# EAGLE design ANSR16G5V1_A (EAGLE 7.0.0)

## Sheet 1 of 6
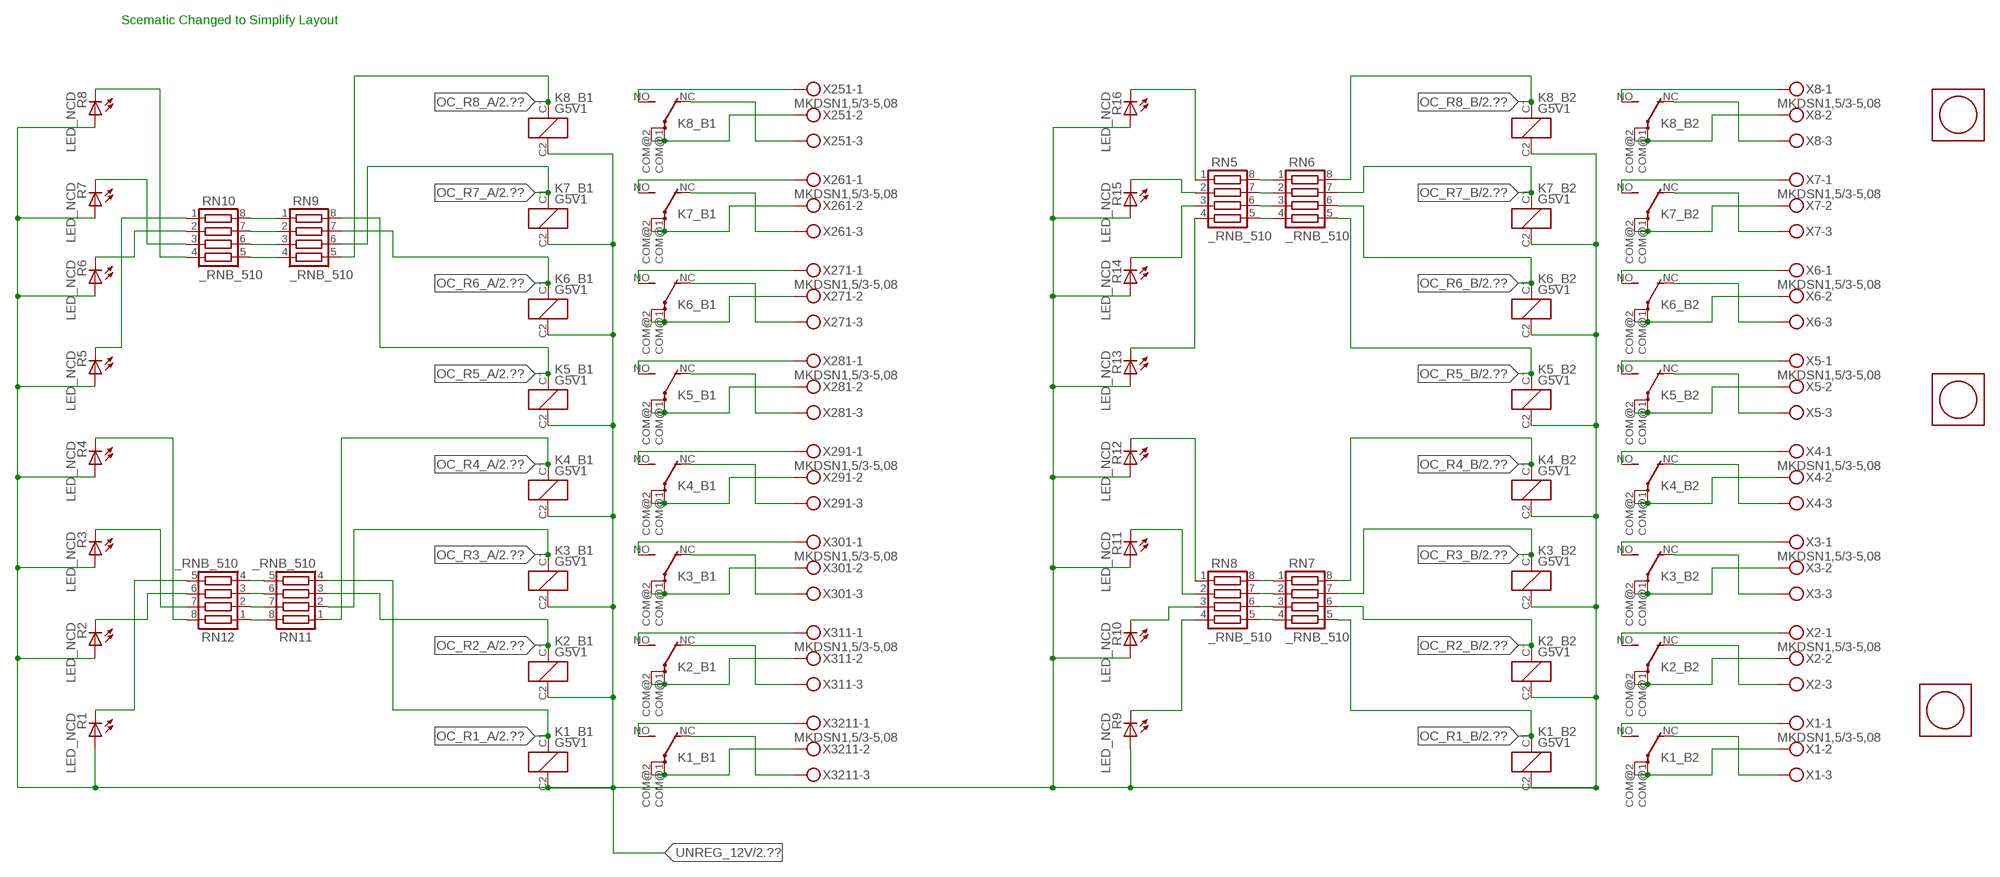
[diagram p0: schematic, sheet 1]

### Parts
K1_B1  G5V1  [G5V1]
K1_B2  G5V1  [G5V1]
K2_B1  G5V1  [G5V1]
K2_B2  G5V1  [G5V1]
K3_B1  G5V1  [G5V1]
K3_B2  G5V1  [G5V1]
K4_B1  G5V1  [G5V1]
K4_B2  G5V1  [G5V1]
K5_B1  G5V1  [G5V1]
K5_B2  G5V1  [G5V1]
K6_B1  G5V1  [G5V1]
K6_B2  G5V1  [G5V1]
K7_B1  G5V1  [G5V1]
K7_B2  G5V1  [G5V1]
K8_B1  G5V1  [G5V1]
K8_B2  G5V1  [G5V1]
R1  LED_NCD  [CHIPLED_0603]
R2  LED_NCD  [CHIPLED_0603]
R3  LED_NCD  [CHIPLED_0603]
R4  LED_NCD  [CHIPLED_0603]
R5  LED_NCD  [CHIPLED_0603]
R6  LED_NCD  [CHIPLED_0603]
R7  LED_NCD  [CHIPLED_0603]
R8  LED_NCD  [CHIPLED_0603]
R9  LED_NCD  [CHIPLED_0603]
R10  LED_NCD  [CHIPLED_0603]
R11  LED_NCD  [CHIPLED_0603]
R12  LED_NCD  [CHIPLED_0603]
R13  LED_NCD  [CHIPLED_0603]
R14  LED_NCD  [CHIPLED_0603]
R15  LED_NCD  [CHIPLED_0603]
R16  LED_NCD  [CHIPLED_0603]
RN5  _RNB_510  [RNB]
RN6  _RNB_510  [RNB]
RN7  _RNB_510  [RNB]
RN8  _RNB_510  [RNB]
RN9  _RNB_510  [RNB]
RN10  _RNB_510  [RNB]
RN11  _RNB_510  [RNB]
RN12  _RNB_510  [RNB]
U$1  PCB_MOUNTING_HOLE  [PCB_MOUNTING_HOLE]
U$2  PCB_MOUNTING_HOLE  [PCB_MOUNTING_HOLE]
U$3  PCB_MOUNTING_HOLE  [PCB_MOUNTING_HOLE]
X1  MKDSN1,5/3-5,08  [MKDSN1,5/3-5,08]
X2  MKDSN1,5/3-5,08  [MKDSN1,5/3-5,08]
X3  MKDSN1,5/3-5,08  [MKDSN1,5/3-5,08]
X4  MKDSN1,5/3-5,08  [MKDSN1,5/3-5,08]
X5  MKDSN1,5/3-5,08  [MKDSN1,5/3-5,08]
X6  MKDSN1,5/3-5,08  [MKDSN1,5/3-5,08]
X7  MKDSN1,5/3-5,08  [MKDSN1,5/3-5,08]
X8  MKDSN1,5/3-5,08  [MKDSN1,5/3-5,08]
X251  MKDSN1,5/3-5,08  [MKDSN1,5/3-5,08]
X261  MKDSN1,5/3-5,08  [MKDSN1,5/3-5,08]
X271  MKDSN1,5/3-5,08  [MKDSN1,5/3-5,08]
X281  MKDSN1,5/3-5,08  [MKDSN1,5/3-5,08]
X291  MKDSN1,5/3-5,08  [MKDSN1,5/3-5,08]
X301  MKDSN1,5/3-5,08  [MKDSN1,5/3-5,08]
X311  MKDSN1,5/3-5,08  [MKDSN1,5/3-5,08]
X3211  MKDSN1,5/3-5,08  [MKDSN1,5/3-5,08]

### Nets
N$1: K8_B2.COM@1(2:P) K8_B2.COM@2(2:P) X8.2
N$2: K8_B2.NC(2:O) X8.3
N$3: K8_B2.NO(2:S) X8.1
N$4: K7_B2.NO(2:S) X7.1
N$5: K6_B2.NO(2:S) X6.1
N$6: K7_B2.NC(2:O) X7.3
N$7: K7_B2.COM@1(2:P) K7_B2.COM@2(2:P) X7.2
N$8: K6_B2.NC(2:O) X6.3
N$10: K4_B2.NO(2:S) X4.1
N$11: K4_B2.NC(2:O) X4.3
N$12: K4_B2.COM@1(2:P) K4_B2.COM@2(2:P) X4.2
N$14: K6_B2.COM@1(2:P) K6_B2.COM@2(2:P) X6.2
N$33: K5_B2.NC(2:O) X5.3
N$34: K5_B2.COM@1(2:P) K5_B2.COM@2(2:P) X5.2
N$35: K5_B2.NO(2:S) X5.1
N$36: K3_B2.NO(2:S) X3.1
N$37: K3_B2.NC(2:O) X3.3
N$38: K3_B2.COM@1(2:P) K3_B2.COM@2(2:P) X3.2
N$39: K2_B2.NO(2:S) X2.1
N$40: K2_B2.NC(2:O) X2.3
N$41: K2_B2.COM@1(2:P) K2_B2.COM@2(2:P) X2.2
N$42: K1_B2.NO(2:S) X1.1
N$43: K1_B2.NC(2:O) X1.3
N$44: K1_B2.COM@1(2:P) K1_B2.COM@2(2:P) X1.2
N$203: K8_B1.COM@1(2:P) K8_B1.COM@2(2:P) X251.2
N$204: K8_B1.NC(2:O) X251.3
N$205: K8_B1.NO(2:S) X251.1
N$206: K7_B1.NO(2:S) X261.1
N$207: K6_B1.NO(2:S) X271.1
N$208: K7_B1.NC(2:O) X261.3
N$209: K7_B1.COM@1(2:P) K7_B1.COM@2(2:P) X261.2
N$210: K6_B1.NC(2:O) X271.3
N$211: K6_B1.COM@1(2:P) K6_B1.COM@2(2:P) X271.2
N$212: K5_B1.NC(2:O) X281.3
N$213: K5_B1.COM@1(2:P) K5_B1.COM@2(2:P) X281.2
N$214: K5_B1.NO(2:S) X281.1
N$215: K4_B1.NO(2:S) X291.1
N$216: K4_B1.NC(2:O) X291.3
N$217: K4_B1.COM@1(2:P) K4_B1.COM@2(2:P) X291.2
N$218: K3_B1.NO(2:S) X301.1
N$219: K3_B1.NC(2:O) X301.3
N$220: K3_B1.COM@1(2:P) K3_B1.COM@2(2:P) X301.2
N$221: K2_B1.NO(2:S) X311.1
N$222: K2_B1.NC(2:O) X311.3
N$223: K2_B1.COM@1(2:P) K2_B1.COM@2(2:P) X311.2
N$224: K1_B1.NO(2:S) X3211.1
N$225: K1_B1.NC(2:O) X3211.3
N$226: K1_B1.COM@1(2:P) K1_B1.COM@2(2:P) X3211.2
N$441: R16.C RN5.1
N$442: RN7.2 RN8.7
N$443: RN7.3 RN8.6
N$444: RN7.4 RN8.5
N$445: R15.C RN5.2
N$447: R13.C RN5.4
N$448: RN5.5 RN6.4
N$449: RN7.1 RN8.8
N$450: R12.C RN8.1
N$451: RN5.6 RN6.3
N$452: R11.C RN8.2
N$453: RN5.7 RN6.2
N$454: RN5.8 RN6.1
N$458: R14.C RN5.3
N$459: R10.C RN8.3
N$463: RN11.5 RN12.4
N$470: R9.C RN8.4
N$473: R1.C RN12.5
N$474: RN11.6 RN12.3
N$475: R2.C RN12.6
N$476: R3.C RN12.7
N$477: RN9.4 RN10.5
N$478: RN9.3 RN10.6
N$479: RN9.2 RN10.7
N$480: RN9.1 RN10.8
N$481: RN11.7 RN12.2
N$482: R5.C RN10.1
N$483: R4.C RN12.8
N$484: R7.C RN10.3
N$485: R8.C RN10.4
N$486: R6.C RN10.2
N$500: RN11.8 RN12.1
OC_R1_A: K1_B1.C1(1:C1) RN11.4 ; also sheet 2
OC_R1_B: K1_B2.C1(1:C1) RN7.5 ; also sheet 2
OC_R2_A: K2_B1.C1(1:C1) RN11.3 ; also sheet 2
OC_R2_B: K2_B2.C1(1:C1) RN7.6 ; also sheet 2
OC_R3_A: K3_B1.C1(1:C1) RN11.2 ; also sheet 2
OC_R3_B: K3_B2.C1(1:C1) RN7.7 ; also sheet 2
OC_R4_A: K4_B1.C1(1:C1) RN11.1 ; also sheet 2
OC_R4_B: K4_B2.C1(1:C1) RN7.8 ; also sheet 2
OC_R5_A: K5_B1.C1(1:C1) RN9.8 ; also sheet 2
OC_R5_B: K5_B2.C1(1:C1) RN6.5 ; also sheet 2
OC_R6_A: K6_B1.C1(1:C1) RN9.7 ; also sheet 2
OC_R6_B: K6_B2.C1(1:C1) RN6.6 ; also sheet 2
OC_R7_A: K7_B1.C1(1:C1) RN9.6 ; also sheet 2
OC_R7_B: K7_B2.C1(1:C1) RN6.7 ; also sheet 2
OC_R8_A: K8_B1.C1(1:C1) RN9.5 ; also sheet 2
OC_R8_B: K8_B2.C1(1:C1) RN6.8 ; also sheet 2
UNREG_12V: K1_B1.C2(1:C2) K1_B2.C2(1:C2) K2_B1.C2(1:C2) K2_B2.C2(1:C2) K3_B1.C2(1:C2) K3_B2.C2(1:C2) K4_B1.C2(1:C2) K4_B2.C2(1:C2) K5_B1.C2(1:C2) K5_B2.C2(1:C2) K6_B1.C2(1:C2) K6_B2.C2(1:C2) K7_B1.C2(1:C2) K7_B2.C2(1:C2) K8_B1.C2(1:C2) K8_B2.C2(1:C2) R1.A R2.A R3.A R4.A R5.A R6.A R7.A R8.A R9.A R10.A R11.A R12.A R13.A R14.A R15.A R16.A ; also sheet 2,3

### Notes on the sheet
- Scematic Changed to Simplify Layout

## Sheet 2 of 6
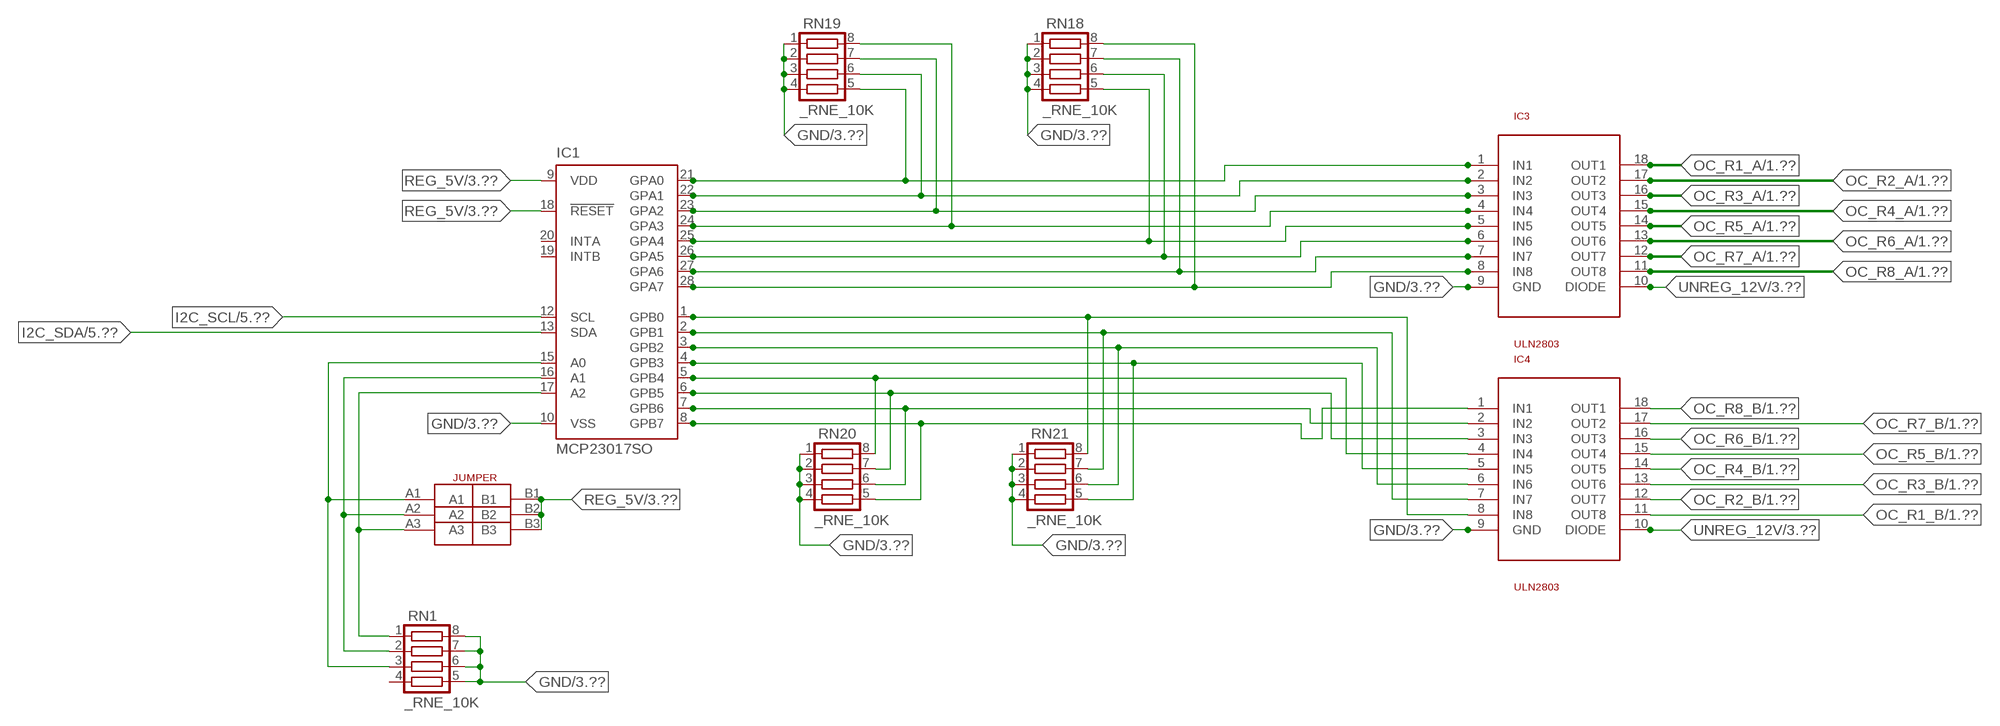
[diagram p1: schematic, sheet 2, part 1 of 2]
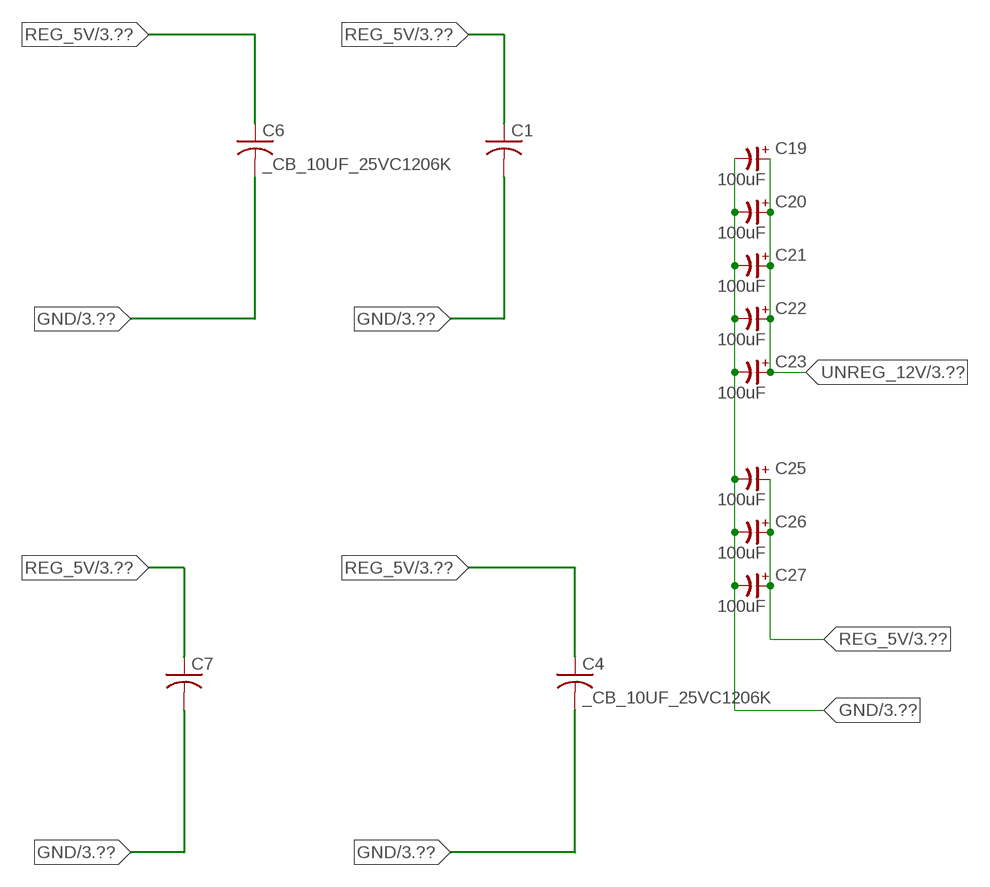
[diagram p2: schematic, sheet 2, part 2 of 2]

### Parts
C1  _CA_.10UF_50VC1206K  [_CA_.1UF_50V]
C4  _CB_10UF_25VC1206K  [_CB_10UF_25V]
C6  _CB_10UF_25VC1206K  [_CB_10UF_25V]
C7  _CA_.10UF_50VC1206K  [_CA_.1UF_50V]
C19  100uF  CP-E-025X060  [E-025X060]
C20  100uF  CP-E-025X060  [E-025X060]
C21  100uF  CP-E-025X060  [E-025X060]
C22  100uF  CP-E-025X060  [E-025X060]
C23  100uF  CP-E-025X060  [E-025X060]
C25  100uF  CP-E-025X060  [E-025X060]
C26  100uF  CP-E-025X060  [E-025X060]
C27  100uF  CP-E-025X060  [E-025X060]
IC1  MCP23017SO  [SO28W]
IC3  ULN2803  [SO18L]
IC4  ULN2803  [SO18L]
JP1  JUMPER_3X2  [JUMPER_3X2]
RN1  _RNE_10K  [RNE]
RN18  _RNE_10K  [RNE]
RN19  _RNE_10K  [RNE]
RN20  _RNE_10K  [RNE]
RN21  _RNE_10K  [RNE]

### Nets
GND: C1.2 C4.2 C6.2 C7.2 C19.- C20.- C21.- C22.- C23.- C25.- C26.- C27.- IC1.10(VSS) IC3.9(GND) IC4.9(GND) RN1.5 RN1.6 RN1.7 RN1.8 RN18.1 RN18.2 RN18.3 RN18.4 RN19.1 RN19.2 RN19.3 RN19.4 RN20.1 RN20.2 RN20.3 RN20.4 RN21.1 RN21.2 RN21.3 RN21.4 ; also sheet 3,4,5,6
I2C_SCL: IC1.12(SCL) ; also sheet 5,6
I2C_SDA: IC1.13(SDA) ; also sheet 5,6
N$78: IC1.15(A0) JP1.A1 RN1.3
N$405: IC1.21(GPA0) IC3.1(IN1) RN19.5
N$406: IC1.25(GPA4) IC3.5(IN5) RN18.5
N$407: IC1.26(GPA5) IC3.6(IN6) RN18.6
N$408: IC1.16(A1) JP1.A2 RN1.2
N$409: IC1.22(GPA1) IC3.2(IN2) RN19.6
N$410: IC1.23(GPA2) IC3.3(IN3) RN19.7
N$411: IC1.24(GPA3) IC3.4(IN4) RN19.8
N$416: IC1.1(GPB0) IC4.8(IN8) RN21.8
N$417: IC1.2(GPB1) IC4.7(IN7) RN21.7
N$418: IC1.3(GPB2) IC4.6(IN6) RN21.6
N$419: IC1.4(GPB3) IC4.5(IN5) RN21.5
N$420: IC1.5(GPB4) IC4.4(IN4) RN20.8
N$421: IC1.6(GPB5) IC4.3(IN3) RN20.7
N$422: IC1.7(GPB6) IC4.2(IN2) RN20.6
N$423: IC1.8(GPB7) IC4.1(IN1) RN20.5
N$498: IC1.17(A2) JP1.A3 RN1.1
N$525: IC1.27(GPA6) IC3.7(IN7) RN18.7
N$526: IC1.28(GPA7) IC3.8(IN8) RN18.8
OC_R1_A: IC3.18(OUT1) ; also sheet 1
OC_R1_B: IC4.11(OUT8) ; also sheet 1
OC_R2_A: IC3.17(OUT2) ; also sheet 1
OC_R2_B: IC4.12(OUT7) ; also sheet 1
OC_R3_A: IC3.16(OUT3) ; also sheet 1
OC_R3_B: IC4.13(OUT6) ; also sheet 1
OC_R4_A: IC3.15(OUT4) ; also sheet 1
OC_R4_B: IC4.14(OUT5) ; also sheet 1
OC_R5_A: IC3.14(OUT5) ; also sheet 1
OC_R5_B: IC4.15(OUT4) ; also sheet 1
OC_R6_A: IC3.13(OUT6) ; also sheet 1
OC_R6_B: IC4.16(OUT3) ; also sheet 1
OC_R7_A: IC3.12(OUT7) ; also sheet 1
OC_R7_B: IC4.17(OUT2) ; also sheet 1
OC_R8_A: IC3.11(OUT8) ; also sheet 1
OC_R8_B: IC4.18(OUT1) ; also sheet 1
REG_5V: C1.1 C4.1 C6.1 C7.1 C25.+ C26.+ C27.+ IC1.9(VDD) IC1.18(!RESET) JP1.B1 JP1.B2 JP1.B3 ; also sheet 3,4,5,6
UNREG_12V: C19.+ C20.+ C21.+ C22.+ C23.+ IC3.10(DIODE) IC4.10(DIODE) ; also sheet 1,3
Unconnected: IC1.19(INTB) IC1.20(INTA) RN1.4

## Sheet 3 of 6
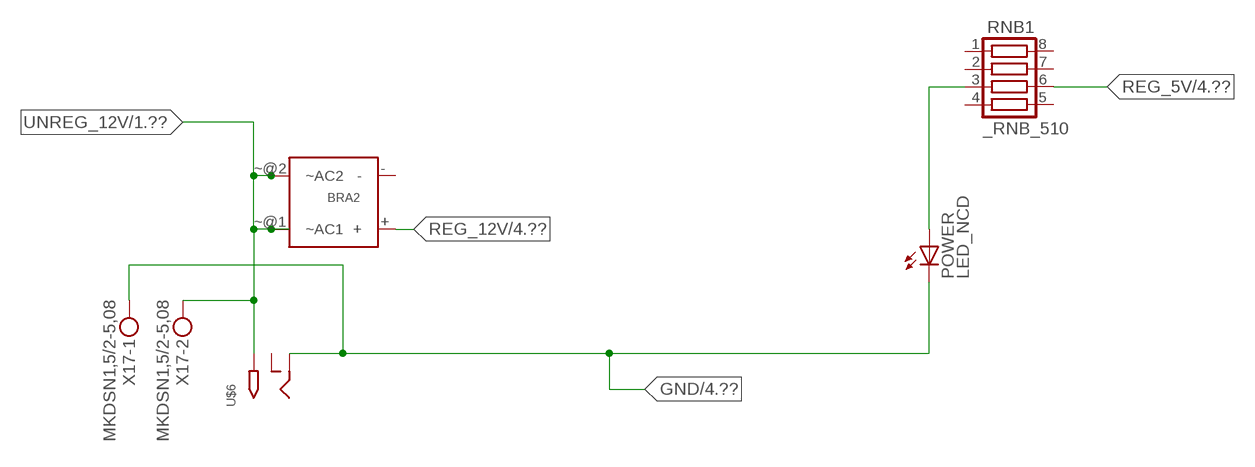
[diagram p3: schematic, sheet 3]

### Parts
BRA2  MB2S_  [MB2S]
POWER  LED_NCD  [CHIPLED_0603]
RNB1  _RNB_510  [RNB]
U$6  2.1MMJACK  [PJ-102A]
X17  MKDSN1,5/2-5,08  [MKDSN1,5/2-5,08]

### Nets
GND: POWER.C U$6.RING X17.1 ; also sheet 2,4,5,6
N$99: POWER.A RNB1.3
REG_5V: RNB1.6 ; also sheet 2,4,5,6
REG_12V: BRA2.+ ; also sheet 4
UNREG_12V: BRA2.~@1(~AC1) BRA2.~@2(~AC2) U$6.TIP X17.2 ; also sheet 1,2
Unconnected: BRA2.- RNB1.1 RNB1.2 RNB1.4 RNB1.5 RNB1.7 RNB1.8 U$6.RING_SW

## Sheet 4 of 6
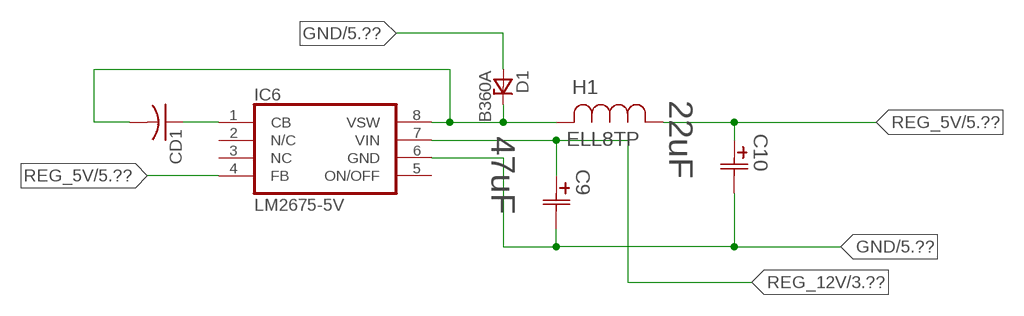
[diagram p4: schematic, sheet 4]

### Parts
C9  47uF  490-5463-6-NDCAP  [C2917(7343)-Y]
C10  22uF  490-5463-6-NDCAP  [C2917(7343)-Y]
CD1  _CD_10NF_50VC1206K  [_CD_10NF_50V]
D1  B360A  [DO214AC_ZENER]
H1  ELL8TP  [IND_ELL8TP]
IC6  LM2675-5V  LM2675  [SO-8]

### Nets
GND: C9.2(C2) C10.2(C2) D1.A IC6.6(GND) ; also sheet 2,3,5,6
N$100: CD1.2 D1.C H1.2 IC6.8(VSW)
N$101: CD1.1 IC6.1(CB)
REG_5V: C10.1(C1) H1.1 IC6.4(FB) ; also sheet 2,3,5,6
REG_12V: C9.1(C1) IC6.7(VIN) ; also sheet 3
Unconnected: IC6.2(N/C) IC6.5(ON/OFF)

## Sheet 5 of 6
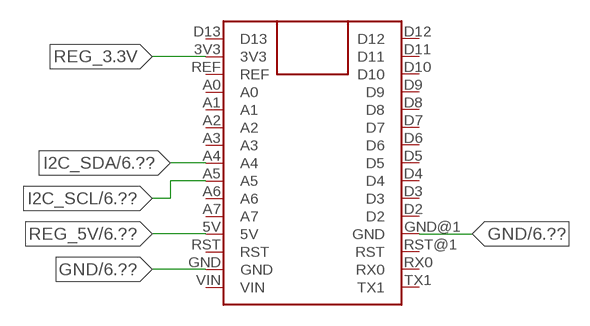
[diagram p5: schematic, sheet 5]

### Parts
FOR_NANO  ARDUINO_NANO  [ARDUINO_NANO]

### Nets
GND: FOR_NANO.GND FOR_NANO.GND@1(GND) ; also sheet 2,3,4,6
I2C_SCL: FOR_NANO.A5 ; also sheet 2,6
I2C_SDA: FOR_NANO.A4 ; also sheet 2,6
REG_3.3V: FOR_NANO.3V3
REG_5V: FOR_NANO.5V ; also sheet 2,3,4,6
Unconnected: FOR_NANO.A0 FOR_NANO.A1 FOR_NANO.A2 FOR_NANO.A3 FOR_NANO.A6 FOR_NANO.A7 FOR_NANO.D2 FOR_NANO.D3 FOR_NANO.D4 FOR_NANO.D5 FOR_NANO.D6 FOR_NANO.D7 FOR_NANO.D8 FOR_NANO.D9 FOR_NANO.D10 FOR_NANO.D11 FOR_NANO.D12 FOR_NANO.D13 FOR_NANO.REF FOR_NANO.RST FOR_NANO.RST@1(RST) FOR_NANO.RX0 FOR_NANO.TX1 FOR_NANO.VIN

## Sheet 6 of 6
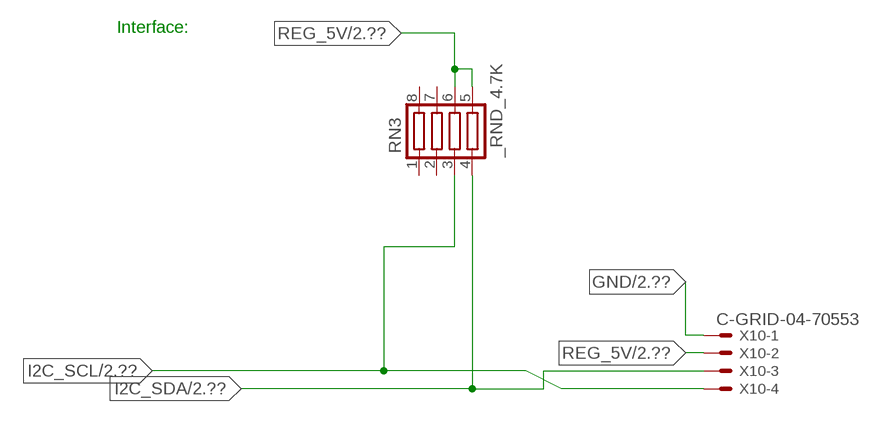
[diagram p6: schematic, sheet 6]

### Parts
RN3  _RND_4.7K  [RND]
X10  C-GRID-04-70553  [70553-04]

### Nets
GND: X10.1 ; also sheet 2,3,4,5
I2C_SCL: RN3.3 X10.4 ; also sheet 2,5
I2C_SDA: RN3.4 X10.3 ; also sheet 2,5
REG_5V: RN3.5 RN3.6 X10.2 ; also sheet 2,3,4,5
Unconnected: RN3.1 RN3.2 RN3.7 RN3.8

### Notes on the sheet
- Interface:

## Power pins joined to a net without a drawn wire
NC: IC6.3(NC)

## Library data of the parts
BRA2 = NCD_ULTIMATE_LIBRARY:MB2S: Bridge Rectifier BRA MB2S 200V 500ma Digikey MB2S-TPMSTR-ND/MB2S-TP
C1 C7 = NCD_ULTIMATE_LIBRARY:_CA_.10UF_50V: Capacitor .1uF SMT
C4 C6 = NCD_ULTIMATE_LIBRARY:_CB_10UF_25V: Capacitor 10uF SMT
C9 C10 = NCD_ULTIMATE_bhaskar:490-5463-6-ND: NCD CAP
C19-C23 C25-C27 = NCD_ULTIMATE_LIBRARY:CP-: Capacitors All Kinds POLARIZED CAP
CD1 = NCD_ULTIMATE_LIBRARY:_CD_10NF_50V: Capacitor 10nF SMT
D1 = NCD_ULTIMATE_bhaskar:B360A: NCD DIODE B350A/B360A
FOR_NANO = NCD_ULTIMATE_CONNECTORS:ARDUINO_NANO
H1 = NCD_ULTIMATE_bhaskar:ELL8TP: NCD coil
IC1 = NCD_ULTIMATE_LIBRARY:MCP23017: Semiconductor Port Expander I/O 16-Bit I2C http://ww1.microchip.com/downloads/en/DeviceDoc/21952a.pdf Source: http://ww1.microchip.com/downloads/en/DeviceDoc/21952a.pdf
IC3 IC4 = NCD_ULTIMATE_LIBRARY:ULN2803: Semiconductor 8 O.C. N-Channel Transistor Driver Digikey ULN2803AFWGCELTR-ND/ULN2803AFWG,C,EL
IC6 = NCD_ULTIMATE_bhaskar:LM2675: LM2675 NCD http://www.ti.com/lit/ds/symlink/lm2675.pdf
JP1 = NCD_ULTIMATE_CONNECTORS:JUMPER_3X2
K1_B1 K1_B2 K2_B1 K2_B2 K3_B1 K3_B2 K4_B1 K4_B2 K5_B1 K5_B2 K6_B1 K6_B2 K7_B1 K7_B2 K8_B1 K8_B2 = NCD_ULTIMATE_LIBRARY:G5V1: RELAY 1 x switch, 0.5 A/125 V AC, 1 A/24 V DC , Omron
POWER R1-R16 = NCD_ULTIMATE_bhaskar:LED_NCD
RN1 RN18-RN21 = NCD_ULTIMATE_LIBRARY:_RNE_10K: Resistor Array RNE SMT 10K x 4 Single Resistor Source: http://www.ctscorp.com/components/Datasheets/CTSChipArrayDs.pdf Digikey 742C083103JPTR-ND/742C083103JP; OC_FARNELL: unknown; OC_NEWARK: unknown
RN3 = NCD_ULTIMATE_LIBRARY:_RND_4.7K: Resistor Array RND SMT 4.7K x 4 Single Resistor Source: http://www.ctscorp.com/components/Datasheets/CTSChipArrayDs.pdf Digikey 742C083472JPTR-ND/742C083472JP; OC_FARNELL: unknown; OC_NEWARK: unknown
RN5-RN12 RNB1 = NCD_ULTIMATE_LIBRARY:_RNB_510: Resistor Array RNB SMT 510 x 4 Single Resistor Source: http://www.ctscorp.com/components/Datasheets/CTSChipArrayDs.pdf Digikey 742C083511JPTR-ND/ 742C083511JP; OC_FARNELL: unknown; OC_NEWARK: unknown
U$1-U$3 = NCD_ULTIMATE_CONNECTORS:PCB_MOUNTING_HOLE
U$6 = NCD_ULTIMATE_CONNECTORS:2.1MMJACK: 2.1mm x 5.5mm DC jack with internal switch. Digikey part #PJ-102A, 4UCON part #05537 By microbuilder.eu
X1-X8 X251 X261 X271 X281 X291 X301 X311 X3211 = NCD_ULTIMATE_CONNECTORS:MKDSN1,5/3-5,08: MKDSN 1,5/ 3-5,08 Printklemme Nennstrom: 13,5 A Nennspannung: 250 V Rastermaß: 5,08 mm Polzahl: 3 Anschlussart: Schraubanschluss Montage: Löten Anschlussrichtung Leiter/Platine: 0 ° Artikelnummer: 1729131 Source: http://eshop.phoenixcontact.com .. 1729131.pdf
X10 = NCD_ULTIMATE_CONNECTORS:C-GRID-04: CONNECTOR 4-Pos I2C wire to board 2.54 mm (0.100") pitch header Digikey WM1342-ND/0015912045; OC_FARNELL: unknown; OC_NEWARK: unknown
X17 = NCD_ULTIMATE_CONNECTORS:MKDSN1,5/2-5,08: MKDSN 1,5/ 2-5,08 Printklemme

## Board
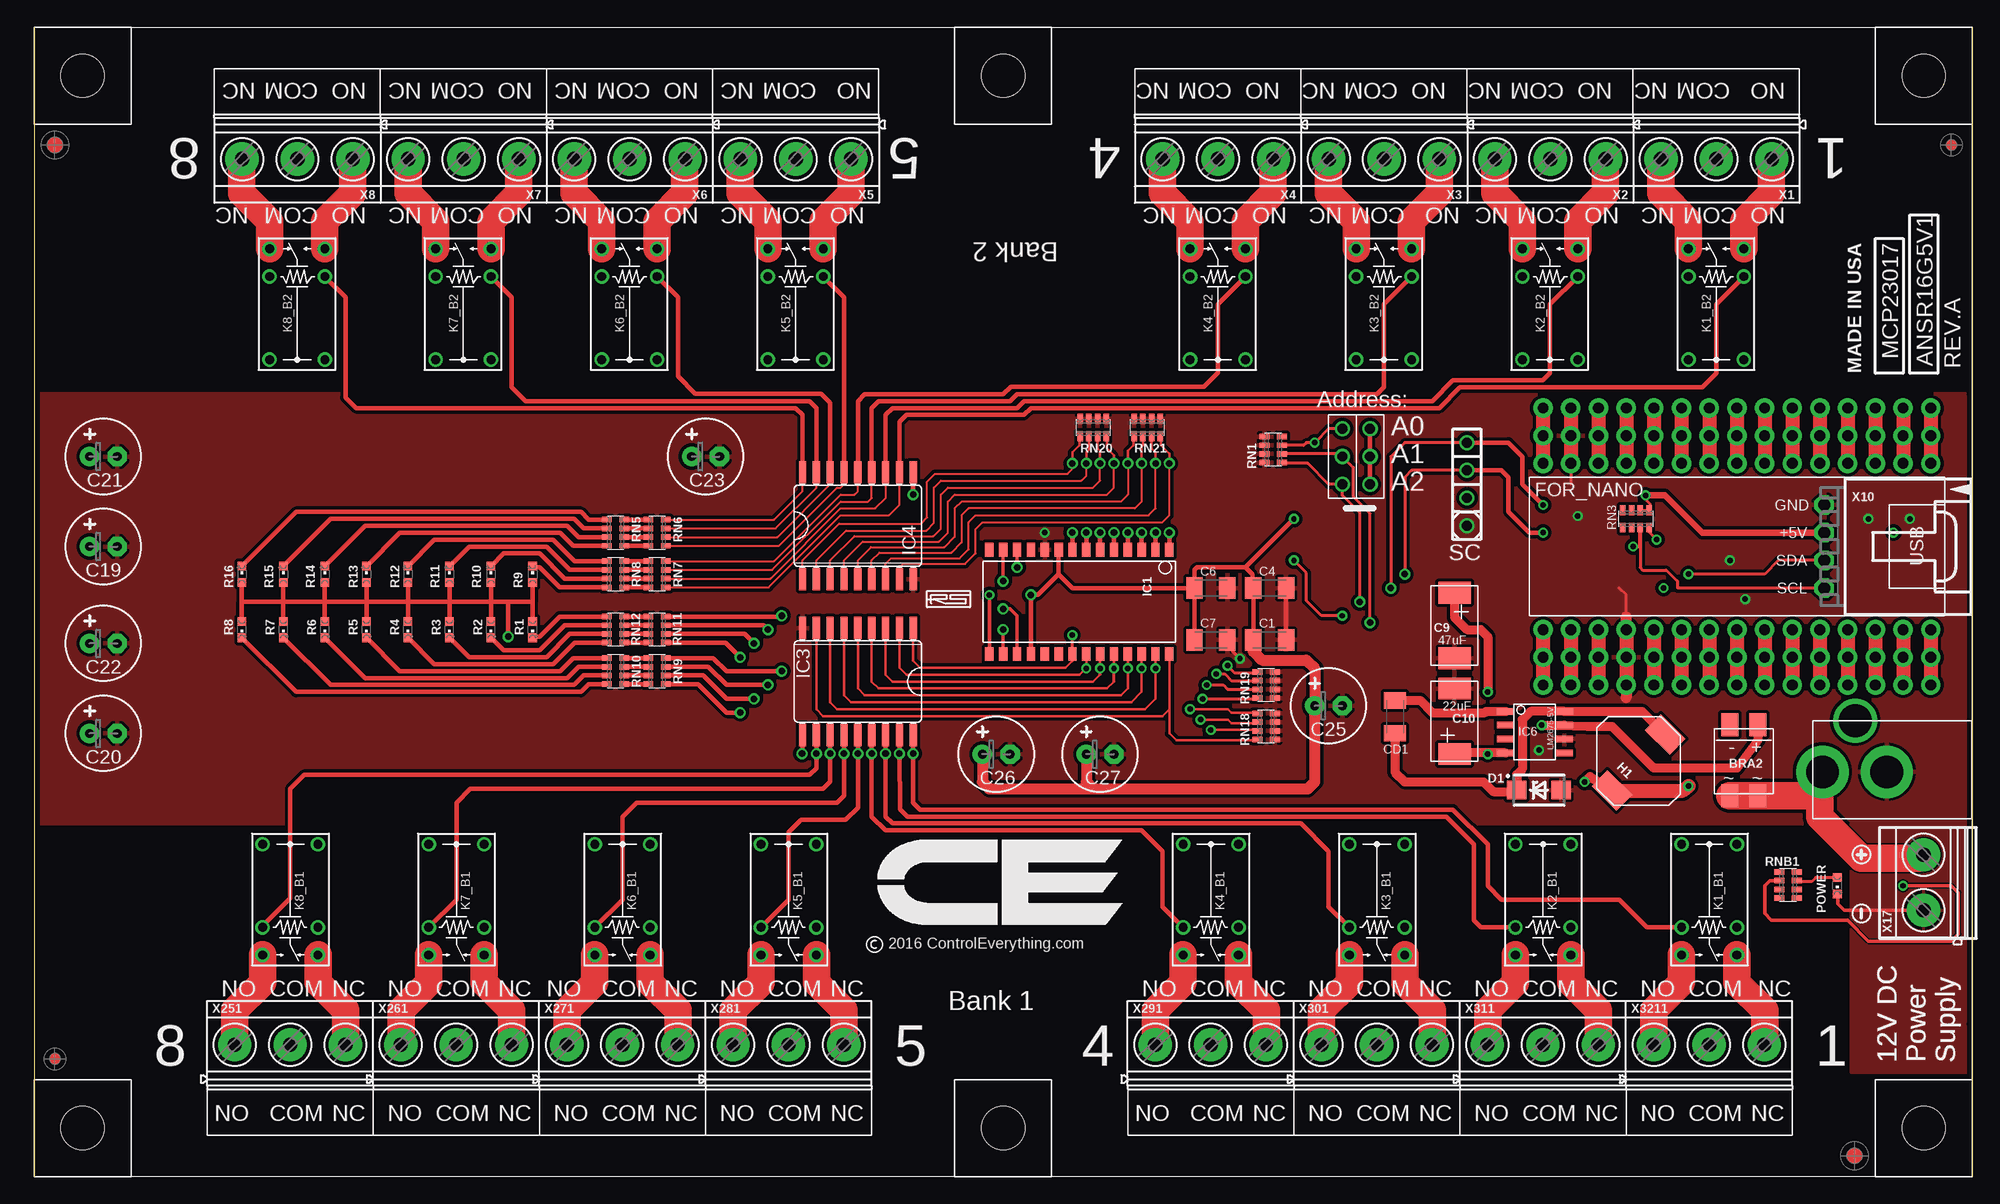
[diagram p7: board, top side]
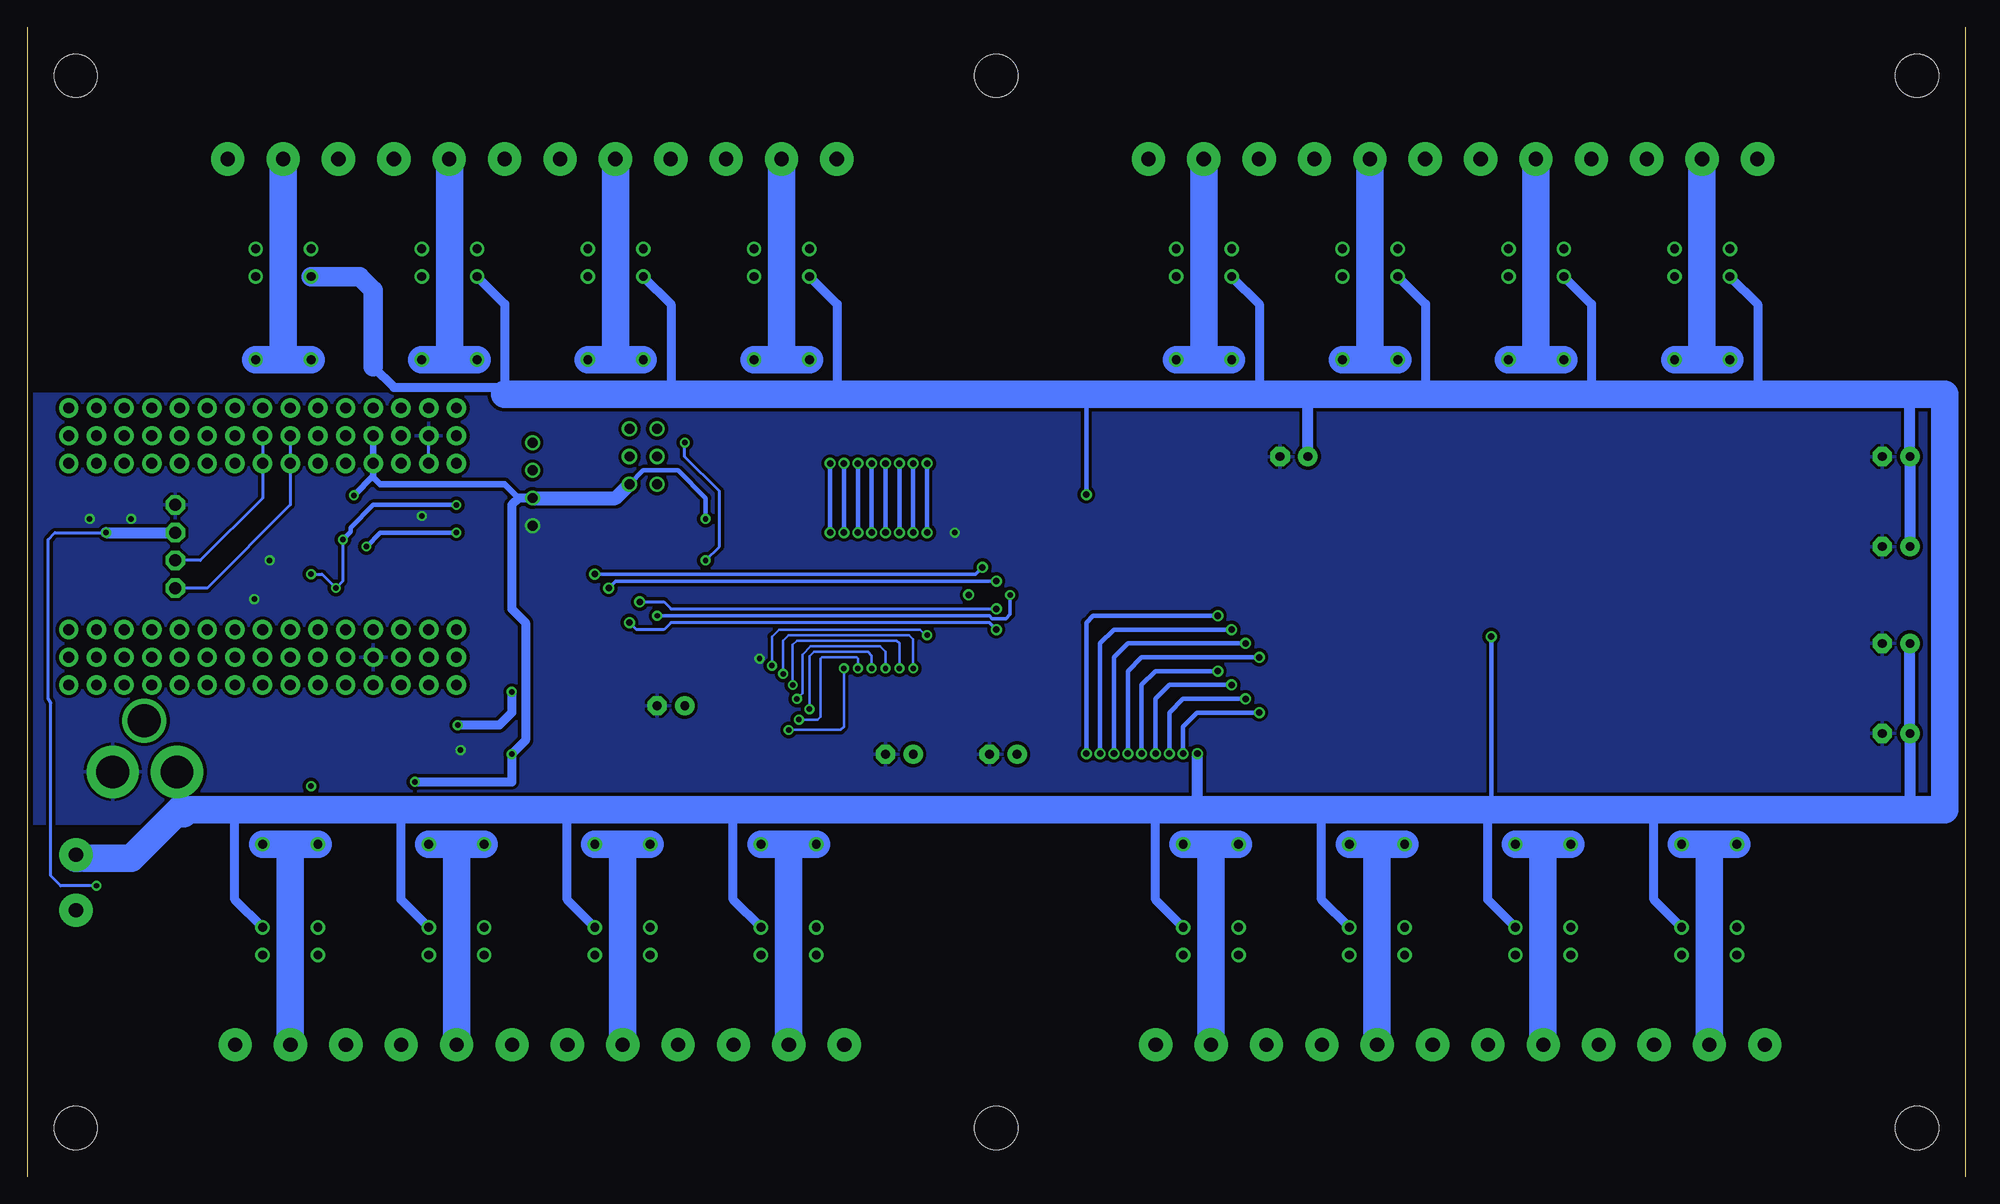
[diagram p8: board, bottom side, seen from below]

Size 177.8 x 105.42 mm. Coordinates in mm from the lower left corner, seen from the top.
Outline: 177.78,105.42 177.78,0
Outline: 0,105.42 0,0.01
Outline: 177.8,71.77 177.8,13.98
Copper layers (1*16): Top 0.035mm / dielectric 1.5mm / Bottom 0.035mm
Design rules "default *": minimum track width 6mil, minimum drill 12mil, track to track 5mil, track to pad 5mil, pad to pad 5mil, via to via 5mil, smd to smd 5mil, copper to edge 20mil, drill to drill 8mil, minimum pad ring 10mil, minimum via ring 8mil, stop-mask expansion 4mil, vias tented up to drill 0mil, thermal gap 10mil

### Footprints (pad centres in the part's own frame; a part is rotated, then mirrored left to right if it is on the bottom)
MB2S = smd 1.55 x 2.1: + 0,-6.5; - 2.54,-6.5; ~@1 0,0; ~@2 2.54,0
_CA_.1UF_50V = smd 1.5 x 2: 1 -1.5,0; 2 1.5,0
_CB_10UF_25V = smd 1.5 x 2: 1 -1.5,0; 2 1.5,0
C2917(7343)-Y = smd 2 x 3: 1 -3,0; 2 3,0
E-025X060 = drill 0.813 pad 1.778: + -1.27,0 | drill 0.813 pad 1.778 octagon: - 1.27,0
_CD_10NF_50V = smd 1.5 x 2: 1 -1.5,0; 2 1.5,0
DO214AC_ZENER = smd 1.8 x 1.7: A 2.05,0; C -2.05,0
ARDUINO_NANO = drill 1 pad 1.778: 3V1 -2.54,-2.54; 3V3 0,-2.54; 5V 0,-27.94; 5V1 -2.54,-27.94; A0 0,-7.62; A1 0,-10.16; A2 0,-12.7; A3 0,-15.24; A4 0,-17.78; A5 0,-20.32; A6 0,-22.86; A7 0,-25.4; A8 -2.54,-7.62; A9 -2.54,-10.16; A10 -2.54,-12.7; A11 -2.54,-15.24; A12 -2.54,-17.78; A13 -2.54,-20.32; A14 -2.54,-22.86; A15 -2.54,-25.4; D1 -2.54,0; D2 20.32,-25.4; D3 20.32,-22.86; D4 20.32,-20.32; D5 20.32,-17.78; D6 20.32,-15.24; D7 20.32,-12.7; D8 20.32,-10.16; D9 20.32,-7.62; D10 20.32,-5.08; D11 20.32,-2.54; D12 20.32,0; D13 0,0; D14 22.86,0; D15 22.86,-2.54; D16 22.86,-5.08; D17 22.86,-7.62; D18 22.86,-10.16; D19 22.86,-12.7; D20 22.86,-15.24; D21 22.86,-17.78; D22 22.86,-20.32; D23 22.86,-22.86; D24 22.86,-25.4; GND 0,-33.02; GND1 -2.54,-33.02; GND@1 20.32,-27.94; GND@2 22.86,-27.94; P$16 2.54,0; P$17 2.54,-2.54; P$18 2.54,-5.08; P$19 2.54,-7.62; P$20 2.54,-10.16; P$21 2.54,-12.7; P$22 2.54,-15.24; P$23 2.54,-17.78; P$24 2.54,-20.32; P$25 2.54,-22.86; P$26 2.54,-25.4; P$27 2.54,-27.94; P$28 2.54,-30.48; P$29 2.54,-33.02; P$30 2.54,-35.56; P$31 17.78,0; P$32 17.78,-2.54; P$33 17.78,-5.08; P$34 17.78,-7.62; P$35 17.78,-10.16; P$36 17.78,-12.7; P$37 17.78,-15.24; P$38 17.78,-17.78; P$39 17.78,-20.32; P$40 17.78,-22.86; P$41 17.78,-25.4; P$42 17.78,-27.94; P$43 17.78,-30.48; P$44 17.78,-33.02; P$45 17.78,-35.56; REF 0,-5.08; REF1 -2.54,-5.08; RST 0,-30.48; RST1 -2.54,-30.48; RST@1 20.32,-30.48; RST@2 22.86,-30.48; RX0 20.32,-33.02; RX1 22.86,-33.02; TX1 20.32,-35.56; TX2 22.86,-35.56; VIN 0,-35.56; VIN1 -2.54,-35.56
IND_ELL8TP = smd 2.054 x 3.2 rotated 45: 1 -2.442,-2.696; 2 2.442,2.442
SO28W = smd 0.762 x 1.27: 1 -7.62,-4.78; 2 -6.35,-4.78; 3 -5.08,-4.78; 4 -3.81,-4.78; 5 -2.54,-4.78; 6 -1.27,-4.78; 7 0,-4.78; 8 1.27,-4.78; 9 2.54,-4.78; 10 3.81,-4.78; 11 5.08,-4.78; 12 6.35,-4.78; 13 7.62,-4.78; 14 8.89,-4.78; 15 8.89,4.78; 16 7.62,4.78; 17 6.35,4.78; 18 5.08,4.78; 19 3.81,4.78; 20 2.54,4.78; 21 1.27,4.78; 22 0,4.78; 23 -1.27,4.78; 24 -2.54,4.78; 25 -3.81,4.78; 26 -5.08,4.78; 27 -6.35,4.78; 28 -7.62,4.78
SO18L = smd 0.66 x 2.032: 1 -5.08,-4.902; 2 -3.81,-4.902; 3 -2.54,-4.902; 4 -1.27,-4.902; 5 0,-4.902; 6 1.27,-4.902; 7 2.54,-4.902; 8 3.81,-4.902; 9 5.08,-4.902; 10 5.08,4.902; 11 3.81,4.902; 12 2.54,4.902; 13 1.27,4.902; 14 0,4.902; 15 -1.27,4.902; 16 -2.54,4.902; 17 -3.81,4.902; 18 -5.08,4.902
SO-8 = smd 0.6 x 1.55: 1 -1.905,-2.69; 2 -0.635,-2.69; 3 0.635,-2.69; 4 1.905,-2.69; 5 1.905,2.71; 6 0.635,2.71; 7 -0.635,2.71; 8 -1.905,2.71
JUMPER_3X2 = drill 0.9: A1 0,5.08; A2 0,2.54; A3 0,0; B1 2.54,5.08; B2 2.54,2.54; B3 2.54,0
G5V1 = drill 0.813: C1 -2.54,2.54; C2 -2.54,-2.54; COM@1 5.08,-2.54; COM@2 5.08,2.54; NC -5.08,-2.54; NO -5.08,2.54
CHIPLED_0603 = smd 0.8 x 0.8: A 0,-0.75; C 0,0.75
RNE = smd 0.5 x 0.9: 1 -1.2,-0.8; 2 -0.4,-0.8; 3 0.4,-0.8; 4 1.2,-0.8; 5 1.2,0.8; 6 0.4,0.8; 7 -0.4,0.8; 8 -1.2,0.8
RND = smd 0.5 x 0.9: 1 -1.2,-0.8; 2 -0.4,-0.8; 3 0.4,-0.8; 4 1.2,-0.8; 5 1.2,0.8; 6 0.4,0.8; 7 -0.4,0.8; 8 -1.2,0.8
RNB = smd 0.5 x 0.9: 1 -1.2,-0.8; 2 -0.4,-0.8; 3 0.4,-0.8; 4 1.2,-0.8; 5 1.2,0.8; 6 0.4,0.8; 7 -0.4,0.8; 8 -1.2,0.8
PCB_MOUNTING_HOLE = hole 3.962: 4.445,4.445
PJ-102A = drill 3 pad 4.8: RING 0.1,-3.39; TIP 0.1,-9.29 | drill 3 pad 3.251: RING_SW -4.6,-6.29
MKDSN1,5/3-5,08 = drill 1.3 pad 3.048: 1 -7.641,0.025; 2 -2.561,0.025; 3 2.519,0.025
70553-04 = drill 1.1 pad 1.778 octagon: 1 -3.81,-7.62; 2 -1.27,-7.62; 3 1.27,-7.62; 4 3.81,-7.62
MKDSN1,5/2-5,08 = drill 1.3 pad 3.048: 1 -2.561,0.025; 2 2.519,0.025

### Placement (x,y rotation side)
BRA2  158.12,34.94 180 top
C1  113.35,49.23 0 top
C4  113.35,53.99 0 top
C6  107.95,53.99 0 top
C7  107.95,49.23 0 top
C9  130.3,50.56 270 top
C10  130.3,41.77 90 top
C19  6.35,57.8 0 top
C20  6.35,40.65 0 top
C21  6.35,66.05 0 top
C22  6.35,48.91 0 top
C23  61.59,66.05 0 top
C25  118.75,43.19 0 top
C26  88.27,38.75 0 top
C27  97.79,38.75 0 top
CD1  124.84,42.18 270 top
D1  138.05,35.45 0 top
FOR_NANO  173.99,67.96 270 top
H1  147.19,38.11 0 top
IC1  96.52,52.72 180 top
IC3  75.56,45.42 180 top
IC4  75.56,59.7 0 top
IC6  137.67,40.78 270 top
JP1  120.02,63.51 0 top
K1_B1  153.67,25.41 90 top
K1_B2  154.31,80.02 270 top
K2_B1  138.43,25.41 90 top
K2_B2  139.06,80.02 270 top
K3_B1  123.19,25.41 90 top
K3_B2  123.83,80.02 270 top
K4_B1  107.95,25.41 90 top
K4_B2  108.58,80.02 270 top
K5_B1  69.22,25.41 90 top
K5_B2  69.85,80.02 270 top
K6_B1  53.98,25.41 90 top
K6_B2  54.61,80.02 270 top
K7_B1  38.73,25.41 90 top
K7_B2  39.37,80.02 270 top
K8_B1  23.5,25.41 90 top
K8_B2  24.13,80.02 270 top
POWER  165.42,26.68 180 top
R1  45.72,50.18 180 top
R2  41.91,50.18 180 top
R3  38.1,50.18 180 top
R4  34.29,50.18 180 top
R5  30.48,50.18 180 top
R6  26.67,50.18 180 top
R7  22.86,50.18 180 top
R8  19.05,50.18 180 top
R9  45.72,55.26 0 top
R10  41.91,55.26 0 top
R11  38.1,55.26 0 top
R12  34.29,55.26 0 top
R13  30.48,55.26 0 top
R14  26.67,55.26 0 top
R15  22.86,55.26 0 top
R16  19.05,55.26 0 top
RN1  113.67,66.69 90 top
RN3  146.94,60.34 0 top
RN5  53.34,59.07 270 top
RN6  57.15,59.07 270 top
RN7  57.15,55.26 270 top
RN8  53.34,55.26 270 top
RN9  57.15,46.37 270 top
RN10  53.34,46.37 270 top
RN11  57.15,50.18 90 top
RN12  53.34,50.18 90 top
RN18  113.03,41.29 90 top
RN19  113.03,45.1 90 top
RN20  97.16,68.72 180 top
RN21  102.11,68.72 180 top
RNB1  160.91,26.75 90 top
U$1  93.34,96.53 90 top
U$2  8.89,96.53 90 top
U$3  177.8,96.53 90 top
U$5  PCB_MOUNTING_HOLE  [PCB_MOUNTING_HOLE]  0,8.9 270 top
U$6  173.35,37.22 270 top
U$8  [ICON_MINUS]  167.64,24.14 90 top
U$9  PCB_MOUNTING_HOLE  [PCB_MOUNTING_HOLE]  8.89,96.53 90 top
U$10  PCB_MOUNTING_HOLE  [PCB_MOUNTING_HOLE]  84.45,8.9 270 top
U$11  PCB_MOUNTING_HOLE  [PCB_MOUNTING_HOLE]  168.91,8.9 270 top
U$12  PCB_MOUNTING_HOLE  [PCB_MOUNTING_HOLE]  0,8.9 270 top
U$13  [ICON_PLUS]  167.64,29.54 0 top
U$15  [VISION_REF15]  167,1.92 90 top
U$17  [ICON_MINUS]  167.64,24.14 90 top
U$18  [VISION_REF10]  175.9,94.63 90 top
U$19  [ICON_PLUS]  167.64,29.54 0 top
U$21  [ICON_USA]  167.64,73.67 90 top
U$22  [ICON_MINUS]  167.64,24.14 90 top
U$23  [VISION_REF15]  1.91,94.63 90 top
U$24  [ICON_PLUS]  167.64,29.54 0 top
U$28  [VISION_REF10]  1.91,10.81 90 top
X1  151.76,93.36 180 top
X2  136.53,93.36 180 top
X3  121.28,93.36 180 top
X4  106.05,93.36 180 top
X5  67.31,93.36 180 top
X6  52.07,93.36 180 top
X7  36.83,93.36 180 top
X8  21.59,93.36 180 top
X10  171.83,57.8 270 top
X17  173.35,27 90 top
X251  26.04,12.08 0 top
X261  41.27,12.08 0 top
X271  56.52,12.08 0 top
X281  71.75,12.08 0 top
X291  110.49,12.08 0 top
X301  125.73,12.08 0 top
X311  140.97,12.08 0 top
X3211  156.21,12.08 0 top

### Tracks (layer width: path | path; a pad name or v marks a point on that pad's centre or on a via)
GND  (via drill 0.5, 0.9)
  Top 0.254: 146.05,51.32 146.05,53.35 145.41,53.99 | FOR_NANO.GND@1 146.05,46.37 | 140.97,70.5 140.97,63.51
  Top 0.305: v110.62,47.51 109.22,48.91 109.22,49 C7.2 | X17.1 166.07,24.44 165.48,25.03 165.48,25.87 POWER.C
  Top 0.406: C1.2 C4.2
  Top 1.016: X10.1 164.06,61.61 | 146.05,43.95 146.05,50.18 146.05,51.32
  Bottom 0.254: 140.97,65.42 FOR_NANO.GND
  other vias: 92.71,59.07 131.44,59.7 168.28,60.34 141.6,60.59 172.09,60.34 155.57,56.53 156.97,52.97 138.05,39.13
  pour Top (isolate 0.305): -7.62,32.4 -7.62,71.77 178.12,71.77 178.12,32.4
  pour Top (isolate 0.305): 178.12,20.33 166.69,20.33 166.69,32.4 178.12,32.4
  pour Bottom (isolate 0.305): -4.45,32.4 -4.45,71.77 177.8,71.77 177.8,32.4
  pour Top (isolate 0.305): 177.48,9.54 166.69,9.54 166.69,32.4 177.48,32.4
  pour Top: 177.48,9.54 166.69,9.54 166.69,32.4 177.48,32.4
I2C_SCL  (via drill 0.5, 0.6, 0.9)
  Top 0.254: v131.44,64.78 126.36,64.78 125.73,64.15 v125.73,55.26 | X10.4 150.75,53.99 150.75,54.62 149.73,55.64 147.57,55.64 147.34,55.87 RN3.3 147.32,59.52 147.32,57.8 v146.69,57.8
  Top 0.305: v90.17,55.89 IC1.12
  Top 0.406: v131.44,64.78 134.62,64.78 135.25,64.15 135.25,60.97 137.16,59.07 v138.43,59.07
  Bottom 0.254: FOR_NANO.A5 153.67,61.61 161.29,53.99 X10.4
  Bottom 0.305: v125.73,55.26 90.81,55.26 v90.17,55.89
  Bottom 0.406: v138.43,59.07 145.41,59.07 v146.69,57.8
I2C_SDA  (via drill 0.5, 0.6, 0.9)
  Top 0.254: v131.44,67.32 125.73,67.32 124.46,66.05 v124.46,53.99 | RN3.4 148.14,59.14 v148.84,58.43 | 149.47,53.98 v149.48,53.99 | X10.3 160.02,56.53 158.75,55.26 v151.76,55.26
  Top 0.305: v88.9,54.62 IC1.13
  Top 0.406: v131.44,67.32 135.25,67.32 136.53,66.05 136.53,63.51 v138.43,61.61
  Bottom 0.254: v148.84,58.43 148.84,54.62 v149.48,53.99 150.75,55.26 v151.76,55.26 | FOR_NANO.A4 156.21,62.24 161.93,56.53 X10.3
  Bottom 0.305: v88.9,54.62 123.83,54.62 v124.46,53.99
  Bottom 0.406: v138.43,61.61 146.07,61.61 RN3.4 148.14,59.14 v148.84,58.43
N$1
  Bottom 2.54: K8_B2.COM@2 24.13,74.94 | 24.13,74.94 K8_B2.COM@1 | X8.2 24.15,74.96 24.13,74.94
N$2
  Top 2.54: K8_B2.NC 21.59,87.64 19.05,90.18 19.05,93.31 X8.3
N$3
  Top 2.54: K8_B2.NO 26.67,87.64 29.21,90.18 29.21,93.31 X8.1
N$4
  Top 2.54: K7_B2.NO 41.91,87.64 44.45,90.18 44.45,93.31 X7.1
N$5
  Top 2.54: K6_B2.NO 57.15,87.64 59.69,90.18 59.69,93.31 X6.1
N$6
  Top 2.54: K7_B2.NC 36.83,87.64 34.29,90.18 34.29,93.31 X7.3
N$7
  Bottom 2.54: K7_B2.COM@2 39.37,74.94 | 39.37,74.94 K7_B2.COM@1 | X7.2 39.39,74.96 39.37,74.94
N$8
  Top 2.54: K6_B2.NC 52.07,87.64 49.53,90.18 49.53,93.31 X6.3
N$10
  Top 2.54: K4_B2.NO 111.12,87.64 113.67,90.18 113.67,93.31 X4.1
N$11
  Top 2.54: K4_B2.NC 106.05,87.64 103.5,90.18 103.5,93.31 X4.3
N$12
  Bottom 2.54: K4_B2.COM@2 108.58,74.94 | 108.58,74.94 K4_B2.COM@1 | X4.2 108.61,74.96 108.58,74.94
N$14
  Bottom 2.54: K6_B2.COM@2 54.61,74.94 | 54.61,74.94 K6_B2.COM@1 | X6.2 54.63,74.96 54.61,74.94
N$33
  Top 2.54: K5_B2.NC 67.31,87.64 64.77,90.18 64.77,93.31 X5.3
N$34
  Bottom 2.54: K5_B2.COM@2 69.85,74.94 | 69.85,74.94 K5_B2.COM@1 | X5.2 69.87,74.96 69.85,74.94
N$35
  Top 2.54: K5_B2.NO 72.39,87.64 74.93,90.18 74.93,93.31 X5.1
N$36
  Top 2.54: K3_B2.NO 126.36,87.64 128.91,90.18 128.91,93.31 X3.1
N$37
  Top 2.54: K3_B2.NC 121.28,87.64 118.75,90.18 118.75,93.31 X3.3
N$38
  Bottom 2.54: 123.83,74.94 K3_B2.COM@1 | K3_B2.COM@2 123.83,74.94 | 123.83,74.94 123.83,93.31 X3.2
N$39
  Top 2.54: K2_B2.NO 141.6,87.64 144.15,90.18 144.15,93.31 X2.1
N$40
  Top 2.54: K2_B2.NC 136.53,87.64 133.99,90.18 133.99,93.31 X2.3
N$41
  Bottom 2.54: 139.06,74.94 K2_B2.COM@1 | K2_B2.COM@2 139.06,74.94 | 139.06,74.94 139.06,93.31 X2.2
N$42
  Top 2.54: K1_B2.NO 156.84,87.64 159.38,90.18 159.38,93.31 X1.1
N$43
  Top 2.54: K1_B2.NC 151.76,87.64 149.22,90.18 149.22,93.31 X1.3
N$44
  Bottom 2.54: K1_B2.COM@1 154.31,74.94 | K1_B2.COM@2 154.31,74.94 | 154.31,74.94 154.31,93.31 X1.2
N$78  (via drill 0.5)
  Top 0.254: v120.02,51.45 118.11,51.45 116.71,52.84 116.71,55.38 v115.57,56.53 | 114.48,67.07 116.46,67.07 116.71,67.32 v117.47,67.32 118.75,68.59 JP1.A1
  Top 0.305: IC1.15 v87.63,53.35 | 114.48,67.07 RN1.3
  Bottom 0.254: v115.57,56.53 114.3,57.8 114.3,62.88 117.47,66.05 v117.47,67.32
  Bottom 0.305: v87.63,53.35 87.63,51.57 88.01,51.19 89.28,51.19 89.53,51.45 v120.02,51.45
N$99
  Top 0.254: POWER.A 163.44,27.43 163.07,27.06 161.79,27.06 RNB1.3
  Top 0.406: 161.75,27.19 RNB1.3
N$100
  Top 0.813: 139.06,42.68 IC6.8 147.5,42.68 H1.2 | 139.06,42.68 137.29,42.68 136.53,41.92 136.53,37.38 136.02,36.87 136.02,35.46 D1.C 135.87,35.32 133.86,35.32 132.97,36.21 125.73,36.21 124.84,37.1 CD1.2 | 139.04,42.71 139.06,42.68
N$101
  Top 0.813: CD1.1 127.15,43.68 128.27,42.56 133.1,42.56 133.22,42.68 IC6.1
N$203
  Bottom 2.54: 23.5,30.49 K8_B1.COM@2 | K8_B1.COM@1 23.5,30.49 | 23.5,30.49 23.5,12.12 X251.2
N$204
  Top 2.54: K8_B1.NC 26.04,17.79 28.57,15.25 28.57,12.12 X251.3
N$205
  Top 2.54: K8_B1.NO 20.95,17.79 18.41,15.25 18.41,12.12 X251.1
N$206
  Top 2.54: K7_B1.NO 36.2,17.79 33.66,15.25 33.66,12.12 X261.1
N$207
  Top 2.54: K6_B1.NO 51.44,17.79 48.9,15.25 48.9,12.12 X271.1
N$208
  Top 2.54: K7_B1.NC 41.27,17.79 43.81,15.25 43.81,12.12 X261.3
N$209
  Bottom 2.54: K7_B1.COM@2 38.73,30.49 | K7_B1.COM@1 38.73,30.49 | 38.73,30.49 38.73,12.12 X261.2
N$210
  Top 2.54: K6_B1.NC 56.52,17.79 59.05,15.25 59.05,12.12 X271.3
N$211
  Bottom 2.54: K6_B1.COM@2 53.98,30.49 | K6_B1.COM@1 53.98,30.49 | 53.98,30.49 53.98,12.12 X271.2
N$212
  Top 2.54: K5_B1.NC 71.75,17.79 74.3,15.25 74.3,12.12 X281.3
N$213
  Bottom 2.54: K5_B1.COM@2 69.22,30.49 | K5_B1.COM@1 69.22,30.49 | 69.22,30.49 69.22,12.12 X281.2
N$214
  Top 2.54: K5_B1.NO 66.67,17.79 64.14,15.25 64.14,12.12 X281.1
N$215
  Top 2.54: K4_B1.NO 105.41,17.79 102.87,15.25 102.87,12.12 X291.1
N$216
  Top 2.54: K4_B1.NC 110.49,17.79 113.03,15.25 113.03,12.12 X291.3
N$217
  Bottom 2.54: 107.95,30.49 K4_B1.COM@2 | K4_B1.COM@1 107.95,30.49 | 107.95,30.49 107.95,12.12 X291.2
N$218
  Top 2.54: K3_B1.NO 120.65,17.79 118.11,15.25 118.11,12.12 X301.1
N$219
  Top 2.54: K3_B1.NC 125.73,17.79 128.27,15.25 128.27,12.12 X301.3
N$220
  Bottom 2.54: 123.19,30.49 K3_B1.COM@2 | K3_B1.COM@1 123.19,30.49 | 123.19,30.49 123.19,12.12 X301.2
N$221
  Top 2.54: K2_B1.NO 135.89,17.79 133.35,15.25 133.35,12.12 X311.1
N$222
  Top 2.54: K2_B1.NC 140.97,17.79 143.51,15.25 143.51,12.12 X311.3
N$223
  Bottom 2.54: 138.43,30.49 K2_B1.COM@2 | K2_B1.COM@1 138.43,30.49 | 138.43,30.49 138.43,12.12 X311.2
N$224
  Top 2.54: K1_B1.NO 151.13,17.79 148.59,15.25 148.59,12.12 X3211.1
N$225
  Top 2.54: K1_B1.NC 156.21,17.79 158.75,15.25 158.75,12.12 X3211.3
N$226
  Bottom 2.54: 153.67,30.49 K1_B1.COM@2 | K1_B1.COM@1 153.67,30.49 | 153.67,30.49 153.67,12.12 X3211.2
N$405  (via drill 0.5)
  Top 0.229: IC1.21 95.25,47.32 94.61,46.68 81.28,46.68 80.64,47.32 IC3.1
  Top 0.254: 95.25,47.32 v95.25,49.67 | v109.47,46.88 110.11,46.24 112.17,46.24
  Top 0.305: 112.17,46.24 112.23,46.24 RN19.5
  Bottom 0.229: v95.25,49.67 95.25,49.54 95.89,50.18 108.84,50.18 109.47,49.54 v109.47,46.88
N$406  (via drill 0.5)
  Top 0.229: IC1.25 v100.34,46.62 100.33,44.78 99.69,44.15 76.2,44.15 75.56,44.78 IC3.5 | v106.05,42.87 109.54,42.87 109.86,42.56 112.16,42.56 RN18.5
  Bottom 0.229: v100.34,46.62 100.33,47.79 100.69,48.15 105.64,48.15 106.05,47.74 v106.05,42.87
N$407  (via drill 0.5)
  Top 0.229: IC1.26 v101.6,46.62 101.6,44.46 100.65,43.51 74.93,43.51 74.3,44.15 IC3.6 | v107,41.92 109.54,41.92 109.86,41.61 112.15,41.61 RN18.6
  Bottom 0.229: v101.6,46.62 101.6,47.51 101.73,47.64 104.9,47.64 105.03,47.51 105.03,42.18 105.28,41.92 v107,41.92
N$408  (via drill 0.6)
  Top 0.254: v122.56,50.81 122.56,60.85 121.03,62.37 121.03,65.04 JP1.A2 119.76,66.05 119.51,66.31 114.48,66.31 RN1.2
  Top 0.305: v88.9,50.18 IC1.16
  Bottom 0.254: 89.53,50.81 118.75,50.81 119.38,50.18 121.92,50.18 v122.56,50.81
  Bottom 0.305: 89.53,50.81 v88.9,50.18
N$409  (via drill 0.5)
  Top 0.229: IC1.22 96.52,46.68 95.89,46.05 80.01,46.05 79.38,46.68 IC3.2
  Top 0.254: 96.52,46.68 v96.52,46.62 | v108.46,46.11 109.22,46.11 109.86,45.48 112.21,45.48 RN19.6
  Bottom 0.229: v96.52,46.62 96.52,49.29 96.9,49.67 107.95,49.67 108.46,49.16 v108.46,46.11
N$410  (via drill 0.5)
  Top 0.229: IC1.23 97.79,46.05 97.16,45.42 78.74,45.42 78.11,46.05 IC3.3
  Top 0.254: 97.79,46.05 v97.79,46.62 | v107.57,45.1 109.09,45.1 109.47,44.72 112.21,44.72 RN19.7
  Bottom 0.229: v97.79,46.62 97.79,48.91 98.04,49.16 107.19,49.16 107.57,48.78 v107.57,45.1
  Bottom 0.254: 107.82,44.97 v107.57,45.1
N$411  (via drill 0.5)
  Top 0.229: IC1.24 99.06,45.42 98.42,44.78 77.47,44.78 76.83,45.42 IC3.4
  Top 0.254: 99.06,45.42 v99.06,46.62 | v107.19,43.83 112.16,43.83 RN19.8
  Bottom 0.229: v99.06,46.62 99.06,48.15 99.57,48.65 105.92,48.65 106.68,47.89 106.68,44.34 v107.19,43.83
N$416  (via drill 0.6)
  Top 0.203: 79.38,55.89 79.69,56.21 85.41,56.21 86.36,57.16 86.36,59.39 87,60.02 103.5,60.02 104.14,60.65 v104.14,65.42
  Top 0.229: v104.14,65.42 104.14,66.31 103.38,67.07 103.38,67.85 RN21.8
  Top 0.406: v104.14,59.07 IC1.1 | IC4.8 79.38,55.89
  Bottom 0.406: v104.14,65.42 v104.14,59.07
N$417  (via drill 0.6)
  Top 0.203: IC4.7 78.11,56.21 78.61,56.72 84.9,56.72 85.72,57.54 85.72,60.02 86.36,60.65 102.23,60.65 102.87,61.29 v102.87,65.42
  Top 0.229: v102.87,65.42 102.87,66.43 102.49,66.81 102.49,67.9 RN21.7
  Top 0.406: v102.87,59.07 IC1.2
  Bottom 0.406: v102.87,65.42 v102.87,59.07
N$418  (via drill 0.6)
  Top 0.203: IC4.6 76.83,56.53 77.53,57.23 84.14,57.23 85.09,58.18 85.09,60.65 85.72,61.29 100.97,61.29 101.6,61.93 v101.6,65.42
  Top 0.229: v101.6,65.42 101.6,66.94 101.73,67.07 101.73,67.9 RN21.6
  Top 0.406: v101.6,59.07 IC1.3
  Bottom 0.406: v101.6,65.42 v101.6,59.07
N$419  (via drill 0.6)
  Top 0.203: IC4.5 75.56,56.53 76.77,57.73 83.5,57.73 84.45,58.69 84.45,61.29 85.09,61.93 99.69,61.93 100.33,62.56 v100.33,65.42
  Top 0.229: v100.33,65.42 100.33,66.56 100.84,67.07 100.84,67.85 RN21.5
  Top 0.406: v100.33,59.07 IC1.4
  Bottom 0.406: v100.33,59.07 v100.33,65.42
N$420  (via drill 0.6)
  Top 0.203: IC4.4 74.3,56.53 76.01,58.24 83,58.24 83.82,59.07 83.82,61.93 84.45,62.56 98.42,62.56 99.06,63.19 v99.06,65.42
  Top 0.229: v99.06,65.42 99.06,66.18 98.42,66.81 98.42,67.85 RN20.8
  Top 0.406: v99.06,59.07 IC1.5
  Bottom 0.406: v99.06,65.42 v99.06,59.07
N$421  (via drill 0.6)
  Top 0.203: IC4.3 73.03,56.53 75.25,58.75 82.49,58.75 83.19,59.45 83.19,62.56 83.82,63.19 97.16,63.19 97.79,63.83 v97.79,65.42
  Top 0.229: v97.79,65.42 97.79,66.56 97.54,66.81 97.54,67.9 RN20.7
  Top 0.406: v97.79,59.07 IC1.6
  Bottom 0.406: v97.79,65.42 v97.79,59.07
N$422  (via drill 0.6)
  Top 0.203: IC4.2 71.75,56.53 74.49,59.26 81.85,59.26 82.55,59.96 82.55,63.19 83.19,63.83 96.07,63.83 96.52,64.28 v96.52,65.42
  Top 0.229: IC1.7 96.52,57.16 | v96.52,65.42 96.52,66.43 96.77,66.69 96.77,67.9 RN20.6
  Top 0.406: 96.52,65.05 v96.52,65.42 | v96.52,59.07 IC1.7
  Bottom 0.406: v96.52,65.42 v96.52,59.07
N$423  (via drill 0.6)
  Top 0.203: IC4.1 70.48,56.53 73.85,59.89 81.34,59.89 81.92,60.46 81.92,63.76 82.62,64.47 94.8,64.47 95.25,64.91 v95.25,65.42
  Top 0.229: v95.25,65.42 95.25,66.43 95.89,67.07 95.89,67.85 RN20.5
  Top 0.406: v95.25,59.07 IC1.8
  Bottom 0.406: v95.25,59.07 v95.25,65.42
N$441
  Top 0.406: RN5.1 50.87,60.27 50.16,60.97 24.02,60.97 R16.C
N$442
  Top 0.406: RN8.7 RN7.2
N$443
  Top 0.406: RN7.3 RN8.6
N$444
  Top 0.406: RN8.5 RN7.4
N$445
  Top 0.406: RN5.2 50.4,59.47 49.53,60.34 27.19,60.34 R15.C
N$447
  Top 0.406: RN5.4 49.46,57.87 48.26,59.07 33.54,59.07 R13.C
N$448
  Top 0.406: RN5.5 RN6.4
N$449
  Top 0.406: RN7.1 RN8.8
N$450
  Top 0.406: RN8.1 49.6,56.46 47.62,58.43 36.72,58.43 R12.C
N$451
  Top 0.406: RN5.6 RN6.3
N$452
  Top 0.406: RN8.2 49.13,55.66 46.99,57.8 39.89,57.8 R11.C
N$453
  Top 0.406: RN6.2 RN5.7
N$454
  Top 0.406: RN5.8 RN6.1
N$458
  Top 0.406: RN5.3 49.93,58.67 48.9,59.7 30.36,59.7 R14.C
N$459
  Top 0.406: RN8.3 48.66,54.86 46.35,57.16 43.06,57.16 R10.C
N$463
  Top 0.406: RN12.4 RN11.5
N$470
  Top 0.406: RN8.4 48.19,54.06 46.35,55.89 45.84,55.89 R9.C
N$473
  Top 0.406: RN12.5 48.19,51.38 46.35,49.54 45.84,49.54 R1.C
N$474
  Top 0.406: RN11.6 RN12.3
N$475
  Top 0.406: RN12.6 48.66,50.58 46.35,48.27 43.06,48.27 R2.C
N$476
  Top 0.406: RN12.7 49.13,49.78 46.99,47.64 39.89,47.64 R3.C
N$477
  Top 0.406: RN9.4 RN10.5
N$478
  Top 0.406: RN10.6 RN9.3
N$479
  Top 0.406: RN9.2 RN10.7
N$480
  Top 0.406: RN10.8 RN9.1
N$481
  Top 0.406: RN12.2 RN11.7
N$482
  Top 0.406: RN10.1 49.46,47.57 48.26,46.37 33.54,46.37 R5.C
N$483
  Top 0.406: RN12.8 49.6,48.98 47.62,47 36.72,47 R4.C
N$484
  Top 0.406: RN10.3 50.4,45.97 49.53,45.1 27.19,45.1 R7.C
N$485
  Top 0.406: RN10.4 50.87,45.17 50.16,44.46 24.02,44.46 R8.C
N$486
  Top 0.406: RN10.2 49.93,46.77 48.9,45.73 30.36,45.73 R6.C
N$498  (via drill 0.6)
  Top 0.254: v121.6,52.72 121.6,60.91 120.02,62.5 JP1.A3 118.75,63.51 116.84,65.42 114.53,65.42 RN1.1
  Top 0.305: IC1.17 90.17,51.45 89.53,52.08 v88.9,52.08
  Bottom 0.254: v121.6,52.72 119.38,52.72 118.75,52.08 v88.9,52.08
N$500
  Top 0.406: RN11.8 RN12.1
N$525  (via drill 0.5)
  Top 0.229: IC3.7 73.03,43.51 73.66,42.87 101.92,42.87 102.87,43.83 v102.87,46.62 IC1.27 | v107.95,40.97 111.68,40.97 RN18.7
  Bottom 0.229: v107.95,40.97 103.19,40.97 102.87,41.29 v102.87,46.62
N$526
  Top 0.229: IC1.28 104.14,42.87 | 104.14,42.87 103.5,42.24 72.39,42.24 71.75,42.87 IC3.8 | 104.14,42.87 104.14,40.65 104.78,40.02 112.16,40.02 RN18.8
OC_R1_A  (via drill 0.6)
  Top 0.406: IC3.18 v80.64,38.81 80.64,34.3 81.28,33.67 130.18,33.67 133.35,30.49 133.35,26.68 134.62,25.41 145.41,25.41 147.96,22.87 K1_B1.C1 | RN11.4 68.51,51.38 v68.58,51.45
  Bottom 0.406: v68.58,51.45 80.01,51.45 80.64,50.81 v80.64,38.81
OC_R1_B
  Top 0.203: RN7.5 67.38,54.06 73.98,60.65 78.42,60.65 79.38,61.61 IC4.11
  Top 0.406: IC4.11 79.38,69.23 80.01,69.86 90.81,69.86 91.44,70.5 128.91,70.5 130.81,72.4 153.03,72.4 154.31,73.67 154.31,80.02 K1_B2.C1
OC_R2_A  (via drill 0.6)
  Top 0.406: RN11.3 66.91,50.58 v67.31,50.18 | IC3.17 v79.38,38.81 79.42,33.7 80.1,33.03 129.54,33.03 132.08,30.49 132.08,23.51 132.72,22.87 K2_B1.C1
  Bottom 0.406: v67.31,50.18 78.11,50.18 79.38,48.91 v79.38,38.81
OC_R2_B
  Top 0.203: IC4.12 78.11,62.24 77.15,61.29 73.98,61.29 67.55,54.86 RN7.6
  Top 0.406: IC4.12 78.11,69.86 78.74,70.5 90.17,70.5 90.81,71.13 128.27,71.13 130.18,73.04 138.43,73.04 139.06,73.67 139.06,80.02 K2_B2.C1
OC_R3_A  (via drill 0.6)
  Top 0.406: RN11.2 65.17,49.78 v66.04,48.91 | IC3.16 v78.11,38.81 78.11,33.03 78.74,32.4 116.2,32.4 118.75,29.86 118.75,24.78 K3_B1.C1
  Bottom 0.406: v66.04,48.91 76.83,48.91 78.11,47.64 v78.11,38.81
OC_R3_B
  Top 0.203: RN7.7 67.71,55.66 73.98,61.93 76.52,61.93 76.83,62.24 IC4.13
  Top 0.406: IC4.13 76.83,70.5 77.47,71.13 89.53,71.13 90.17,71.77 123.19,71.77 123.83,72.4 123.83,80.02 K3_B2.C1
OC_R4_A  (via drill 0.6)
  Top 0.406: RN11.1 63.43,48.98 v64.77,47.64 | IC3.15 v76.83,38.81 76.83,33.03 78.11,31.76 101.6,31.76 103.5,29.86 103.5,24.78 K4_B1.C1
  Bottom 0.406: v64.77,47.64 75.56,47.64 76.83,46.37 v76.83,38.81
OC_R4_B
  Top 0.203: RN7.8 67.88,56.46 73.98,62.56 75.25,62.56 75.56,62.88 IC4.14
  Top 0.406: IC4.14 75.56,71.13 76.2,71.77 88.9,71.77 89.6,72.47 107.31,72.47 108.58,73.74 108.58,80.02 K4_B2.C1
OC_R5_A  (via drill 0.6)
  Top 0.406: RN9.8 62.3,47.57 63.5,46.37 v68.58,46.37 | IC3.14 v75.56,38.81 75.56,33.86 74.42,32.72 70.36,32.72 69.22,31.57 69.22,25.41 K5_B1.C1
  Bottom 0.406: v68.58,46.37 74.3,46.37 75.56,45.1 v75.56,38.81
OC_R5_B
  Top 0.203: IC4.15 74.3,63.51 73.98,63.19 73.66,63.19 68.33,57.87 RN6.5
  Top 0.406: K5_B2.C1 74.3,80.66 IC4.15
OC_R6_A  (via drill 0.6)
  Top 0.406: RN9.7 61.83,46.77 63.5,45.1 v67.31,45.1 | IC3.13 v74.3,38.81 74.3,34.94 73.66,34.3 55.24,34.3 53.98,33.03 53.98,25.41 K6_B1.C1
  Bottom 0.406: v67.31,45.1 73.03,45.1 74.3,43.83 v74.3,38.81
OC_R6_B
  Top 0.203: RN6.6 68.18,58.67 73.03,63.51 IC4.16
  Top 0.406: IC4.16 73.03,71.01 72.2,71.83 60.62,71.83 59.05,73.4 59.05,80.66 K6_B2.C1
OC_R7_A  (via drill 0.6)
  Top 0.406: RN9.6 61.36,45.97 63.5,43.83 v66.04,43.83 | IC3.12 v73.03,38.81 73.03,36.21 72.39,35.57 40.01,35.57 38.73,34.3 38.73,25.41 K7_B1.C1
  Bottom 0.406: v66.04,43.83 71.75,43.83 73.03,42.56 v73.03,38.81
OC_R7_B
  Top 0.203: RN6.7 68.03,59.47 71.75,63.19 IC4.17
  Top 0.406: IC4.17 71.75,70.5 71.12,71.13 45.09,71.13 43.81,72.4 43.81,80.66 K7_B2.C1
OC_R8_A  (via drill 0.6)
  Top 0.406: RN9.5 60.89,45.17 63.5,42.56 v64.77,42.56 | IC3.11 v71.75,38.81 71.75,37.48 71.12,36.84 24.77,36.84 23.5,35.57 23.5,25.54 20.95,23 K8_B1.C1
  Bottom 0.406: v64.77,42.56 70.48,42.56 71.75,41.29 v71.75,38.81
OC_R8_B
  Top 0.203: RN6.8 67.88,60.27 70.48,62.88 IC4.18
  Top 0.406: IC4.18 70.48,69.86 69.85,70.5 29.53,70.5 28.57,71.45 28.57,80.66 K8_B2.C1
REG_5V  (via drill 0.5, 0.6, 0.9)
  Top 0.254: 122.73,63.34 JP1.B3 | RN3.6 RN3.5 148.21,61.21 148.21,61.73 147.83,62.12 v147.83,62.5
  Top 0.305: 160.06,27.19 RNB1.6 159.21,27.15 158.75,26.68 158.75,24.14 159.38,23.51 166.37,23.51 168.28,21.6 175.9,21.6 176.53,22.24 176.53,26.05 175.9,26.68 v171.45,26.68
  Top 0.406: C1.1 C4.1 111.76,54.07 111.76,55.26 111.12,55.89 | C6.1 C7.1 | JP1.B3 JP1.B2 JP1.B1 | 115.64,60.27 v115.57,60.34 111.12,55.89 | IC1.18 v91.44,53.35 92.08,53.35 93.98,55.26 | 93.98,55.26 IC1.9 | 93.98,55.26 95.25,53.99 C6.1 | C6.1 106.45,55.66 106.68,55.89 111.12,55.89
  Top 0.61: v147.83,62.5 149.61,62.5 153.03,59.07 X10.2
  Top 0.813: H1.1 142.72,36.69 v142.24,36.21 | IC6.4 133.48,38.87 | 133.48,38.87 v133.35,38.75 | 133.48,38.87 130.41,38.87 C10.1
  Top 1.016: C1.1 111.85,48.18 112.65,47.38 116.71,47.38 117.47,46.62 C25.+ 117.47,36.21 116.84,35.57 97.16,35.57 | C27.+ 96.52,36.21 97.16,35.57 | C26.+ 87,36.21 87.63,35.57 97.16,35.57
  Top 1.27: H1.1 151.23,35.42 v151.76,35.83
  Bottom 0.254: v171.45,26.68 174.74,26.68 175.64,27.58 175.64,43.45 175.9,43.83 175.9,58.43 175.26,59.07 v170.56,59.07
  Bottom 0.406: v115.57,60.34 115.57,62.24 118.11,64.78 121.28,64.78 JP1.B3
  Bottom 0.61: FOR_NANO.5V 146.05,64.27 | 146.05,64.27 v147.83,62.5 | 146.05,64.27 146.05,64.15 145.41,63.51 133.99,63.51 132.72,62.24
  Bottom 0.813: v142.24,36.21 133.35,36.21 v133.35,38.75 132.08,40.02 132.08,50.81 133.35,52.08 133.35,61.61 132.72,62.24 v131.44,62.24
  Bottom 1.016: v170.56,59.07 X10.2
  Bottom 1.27: v131.44,62.24 123.83,62.24 JP1.B3
REG_12V  (via drill 0.5)
  Top 0.813: BRA2.+ 158.12,40.02 156.21,37.48 148.59,37.48 144.78,41.29 142.49,41.29 v138.3,41.41 IC6.7 | C9.1 130.3,51.32 131.44,50.18 132.72,50.18 133.35,49.54 v133.35,44.46
  Bottom 0.813: v133.35,44.46 133.35,42.56 134.49,41.41 v138.3,41.41
UNREG_12V  (via drill 0.6)
  Top 0.305: 45.72,52.72 R1.A
  Top 0.406: IC4.10 v80.64,62.56 | R8.A 19.05,52.72 | R15.A 22.86,52.72 | R6.A 26.67,52.72 | 30.48,52.72 R13.A | R4.A 34.29,52.72 | R3.A 38.1,52.72 | R2.A 41.91,52.72 | R16.A 19.05,52.72 | 19.05,52.72 22.86,52.72 | R7.A 22.86,52.72 | 22.86,52.72 26.67,52.72 | R14.A 26.67,52.72 | 26.67,52.72 30.48,52.72 | R5.A 30.48,52.72 | 30.48,52.72 34.29,52.72 | R12.A 34.29,52.72 | 34.29,52.72 38.1,52.72 | R11.A 38.1,52.72 | 38.1,52.72 41.91,52.72 | R10.A 41.91,52.72 | R9.A 45.72,52.72 | 45.72,50.81 45.72,52.72 | 45.72,52.72 43.5,52.72 | 41.91,52.72 43.5,52.72 | 43.5,52.72 v43.5,49.54 | IC3.10 70.48,39.38 v70.45,38.81
  Top 2.54: BRA2.~@2 BRA2.~@1 162.51,34.94 U$6.TIP 163.83,36.89 163.83,33.03 167.64,29.22 173.03,29.22 X17.2
  Bottom 0.406: v80.64,62.56 80.64,71.13 80.01,71.77 | v43.5,49.54 43.5,33.67 | 60.39,33.98 60.71,33.67
  Bottom 0.61: 134.62,72.4 133.99,71.77 | 173.35,29.22 173.35,29.49 X17.2
  Bottom 0.813: K8_B1.C2 28.57,25.41 28.57,33.67 | K7_B1.C2 43.81,25.41 43.81,33.67 | K6_B1.C2 59.05,25.41 59.05,33.67 | K5_B1.C2 74.3,25.41 74.3,33.67 | K4_B1.C2 113.03,25.41 113.03,33.67 | K3_B1.C2 128.27,25.41 128.27,33.67 | K2_B1.C2 143.51,25.41 143.51,33.67 | K1_B1.C2 158.75,25.41 158.75,33.67 | K2_B2.C2 133.99,80.02 133.99,71.77 | K3_B2.C2 118.75,80.02 118.75,71.77 | K4_B2.C2 103.5,80.02 103.5,71.77 | K5_B2.C2 64.77,80.02 64.77,71.77 | K6_B2.C2 49.53,80.02 49.53,71.77 | K7_B2.C2 34.29,80.02 34.29,71.77 | K8_B2.C2 19.05,80.02 19.05,71.77 | 146.05,74.31 144.15,72.4 134.62,72.4
  Bottom 1.016: 60.39,33.98 70.45,33.98 v70.45,38.81 | 61.59,71.13 60.96,71.77 | 2.54,34.3 1.91,33.67 | C23.+ 60.33,71.77 | C22.+ C20.+ 5.08,33.67 | C19.+ C21.+ 5.08,71.77
  Bottom 1.778: 146.05,74.31 146.05,81.29 147.32,82.56 K1_B2.C2
  Bottom 2.54: 163.45,33.29 163.83,33.67 | 163.83,33.67 158.75,33.67 143.51,33.67 128.27,33.67 113.03,33.67 74.3,33.67 60.71,33.67 59.05,33.67 43.81,33.67 43.5,33.67 28.57,33.67 5.08,33.67 1.91,33.67 1.91,71.77 5.08,71.77 19.05,71.77 34.29,71.77 49.53,71.77 60.33,71.77 60.96,71.77 64.77,71.77 80.01,71.77 103.5,71.77 118.75,71.77 133.99,71.77 | 173.35,29.22 168.28,29.22 163.83,33.67

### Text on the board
tNames: NC | COM | NO | NC | COM | NO | NC | COM | NO | NC | COM | NO | NC | COM | NO | NC | COM | NO | NC | COM | NO | NC | COM | NO | 8 | 5 | 4 | 1 | NC | COM | NO | NC | COM | NO | NC | COM | NO | NC | COM | NO | NC | COM | NO | NC | COM | NO | NC | COM | NO | NC | COM | NO | ANSR16G5V1 | Bank 2 | MCP23017 | REV.A | Address: | A0 | A1 | A2 | GND | +5V | SC | SDA | SCL | 2016 ControlEverything.com | NO | COM | NC | NO | COM | NC | NO | COM | NC | NO | COM | NC | NO | COM | NC | NO | COM | NC | NO | COM | NC | NO | COM | NC | Bank 1 | 8 | 5 | 4 | 1 | 12V DC / Power / Supply | 12V DC / Power / Supply | 12V DC / Power / Supply | NO | COM | NC | NO | COM | NC | NO | COM | NC | NO | COM | NC | NO | COM | NC | NO | COM | NC | NO | COM | NC | NO | COM | NC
